DATA_BLOCK DB 701
TITLE = Data to be transmitted to Kongsberg System
VERSION : 0.1


  STRUCT
   PacketNo1 : BYTE ;	// *** TELEGRAM 1 ***   Block 1 (4 Bytes)
   TelegramNo1 : BYTE ;
   TelegramLength1 : WORD ;	//Block 1 End (4 Bytes)
   DG_1_OVERSPEED_TRIP : BOOL ;	//Block 2 (64 Bytes)
   DG_1_FUEL_OIL_PRESSURE : BOOL ;
   DG_1_INJ_FO_PIPE_LEAK_A : BOOL ;
   DG_1_INJ_FO_PIPE_LEAK_B : BOOL ;
   DG_1_LUBE_OIL_LEVEL : BOOL ;
   DG_1_LO_FLT_DIFF_PR : BOOL ;
   DG_1_FO_FLT_DIFF_PR : BOOL ;
   Spare_1_4_7 : BOOL ;
   DG_1_RUNNING : BOOL ;
   DG_1_START_AIR_PRESSURE : BOOL ;
   DG_1_SYMMETRIZATION : BOOL ;
   Spare_1_5_3 : BOOL ;
   Spare_1_5_4 : BOOL ;
   Spare_1_5_5 : BOOL ;
   Spare_1_5_6 : BOOL ;
   Spare_1_5_7 : BOOL ;
   Spare_1_6_0 : BOOL ;
   Spare_1_6_1 : BOOL ;
   Spare_1_6_2 : BOOL ;
   Spare_1_6_3 : BOOL ;
   Spare_1_6_4 : BOOL ;
   Spare_1_6_5 : BOOL ;
   Spare_1_6_6 : BOOL ;
   Spare_1_6_7 : BOOL ;
   Spare_1_7_0 : BOOL ;
   Spare_1_7_1 : BOOL ;
   Spare_1_7_2 : BOOL ;
   Spare_1_7_3 : BOOL ;
   Spare_1_7_4 : BOOL ;
   Spare_1_7_5 : BOOL ;
   Spare_1_7_6 : BOOL ;
   Spare_1_7_7 : BOOL ;
   DG_1_LO_PRESSURE : INT ;
   DG_1_FUEL_OIL_PRESSUREA : INT ;
   DG_1_HT_CW_PRESSURE : INT ;
   DG_1_CA_PRESSURE : INT ;
   DG_1_INJ_COOL_OIL_PRESS : INT ;
   DG_1_RPM : INT ;
   DG_1_TURBO_CHARGER_A_RPM : INT ;
   DG_1_TURBO_CHARGER_B_RPM : INT ;
   DG_1_LO_TEMP : INT ;
   DG_1_COOL_WATER_TEMP : INT ;
   DG_1_CHARG_AIR_TEMP : INT ;
   DG_1_INJ_COOL_OIL_TEMP : INT ;
   DG_1_EXH_GAS_CYL_01_TEMP : INT ;
   DG_1_EXH_GAS_CYL_02_TEMP : INT ;
   DG_1_EXH_GAS_CYL_03_TEMP : INT ;
   DG_1_EXH_GAS_CYL_04_TEMP : INT ;
   DG_1_EXH_GAS_CYL_05_TEMP : INT ;
   DG_1_EXH_GAS_CYL_06_TEMP : INT ;
   DG_1_EXH_GAS_CYL_07_TEMP : INT ;
   DG_1_EXH_GAS_CYL_08_TEMP : INT ;
   DG_1_EXH_GAS_CYL_09_TEMP : INT ;
   DG_1_EXH_GAS_CYL_10_TEMP : INT ;
   DG_1_EXH_GAS_CYL_11_TEMP : INT ;
   DG_1_EXH_GAS_CYL_12_TEMP : INT ;
   DG_1_EXH_GAS_CYL_13_TEMP : INT ;
   DG_1_EXH_GAS_CYL_14_TEMP : INT ;
   DG_1_EXH_GAS_CYL_15_TEMP : INT ;
   DG_1_EXH_GAS_CYL_16_TEMP : INT ;
   DG_1_EXH_CYL_TEMP_MEAN : INT ;
   DG_1_EXH_GAS_TEMP_COMP : INT ;	//Block 2 End (64 Bytes)
   DG_2_OVERSPEED_TRIP : BOOL ;	//Block 3 (64 Bytes)
   DG_2_FUEL_OIL_PRES : BOOL ;
   DG_2_INJ_FO_PIPE_LEAK_A : BOOL ;
   DG_2_INJ_FO_PIPE_LEAK_B : BOOL ;
   DG_2_ENGINE_LUBE_OIL_LVL : BOOL ;
   DG_2_LO_FLT_DIFF_PR : BOOL ;
   DG_2_FO_FLT_DIFF_PR : BOOL ;
   Spare_1_68_7 : BOOL ;
   DG_2_ENGINE_RUNNING : BOOL ;
   DG_2_START_AIR_PRESSURE : BOOL ;
   DG_2_SYMMETRIZATION : BOOL ;
   Spare_1_69_3 : BOOL ;
   Spare_1_69_4 : BOOL ;
   Spare_1_69_5 : BOOL ;
   Spare_1_69_6 : BOOL ;
   Spare_1_69_7 : BOOL ;
   Spare_1_70_0 : BOOL ;
   Spare_1_70_1 : BOOL ;
   Spare_1_70_2 : BOOL ;
   Spare_1_70_3 : BOOL ;
   Spare_1_70_4 : BOOL ;
   Spare_1_70_5 : BOOL ;
   Spare_1_70_6 : BOOL ;
   Spare_1_70_7 : BOOL ;
   Spare_1_71_0 : BOOL ;
   Spare_1_71_1 : BOOL ;
   Spare_1_71_2 : BOOL ;
   Spare_1_71_3 : BOOL ;
   Spare_1_71_4 : BOOL ;
   Spare_1_71_5 : BOOL ;
   Spare_1_71_6 : BOOL ;
   Spare_1_71_7 : BOOL ;
   DG_2_ENGINE_LO_PRESSURE : INT ;
   DG_2_FUEL_OIL_PRESA : INT ;
   DG_2_HT_CW_PRESSURE : INT ;
   DG_2_CA_PRESSURE : INT ;
   DG_2_INJ_COOL_OIL_PRESS : INT ;
   DG_2_ENGINE_RPM : INT ;
   DG_2_TURBO_CHARGER_A_RPM : INT ;
   DG_2_TURBO_CHARGER_B_RPM : INT ;
   DG_2_ENGINE_LO_TEMP : INT ;
   DG_2_COOL_WATER_TEMP : INT ;
   DG_2_CHARG_AIR_TEMP : INT ;
   DG_2_INJ_COOL_OIL_TEMP : INT ;
   DG_2_EXH_GAS_CYL_01_TEMP : INT ;
   DG_2_EXH_GAS_CYL_02_TEMP : INT ;
   DG_2_EXH_GAS_CYL_03_TEMP : INT ;
   DG_2_EXH_GAS_CYL_04_TEMP : INT ;
   DG_2_EXH_GAS_CYL_05_TEMP : INT ;
   DG_2_EXH_GAS_CYL_06_TEMP : INT ;
   DG_2_EXH_GAS_CYL_07_TEMP : INT ;
   DG_2_EXH_GAS_CYL_08_TEMP : INT ;
   DG_2_EXH_GAS_CYL_09_TEMP : INT ;
   DG_2_EXH_GAS_CYL_10_TEMP : INT ;
   DG_2_EXH_GAS_CYL_11_TEMP : INT ;
   DG_2_EXH_GAS_CYL_12_TEMP : INT ;
   DG_2_EXH_GAS_CYL_13_TEMP : INT ;
   DG_2_EXH_GAS_CYL_14_TEMP : INT ;
   DG_2_EXH_GAS_CYL_15_TEMP : INT ;
   DG_2_EXH_GAS_CYL_16_TEMP : INT ;
   DG_2_EXH_CYL_TEMP_MEAN : INT ;
   DG_2_EXH_GAS_TEMP_COMP : INT ;	//Block 3 End (64 Bytes)
   GEN_1_VOLTAGE_L1_L2 : INT ;	//Block 4 (32 Bytes)
   GEN_1_VOLTAGE_L1_L3 : INT ;
   GEN_1_VOLTAGE_L2_L3 : INT ;
   GEN_1_CURRENT_L1_L2 : INT ;
   GEN_1_CURRENT_L1_L3 : INT ;
   GEN_1_CURRENT_L2_L3 : INT ;
   GEN_1_ACTIVE_POWER : INT ;
   GEN_1_POWER_FACTOR : INT ;
   GEN_1_REACTIVE_POWER : INT ;
   GEN_1_WDG_TEMP_L1 : INT ;
   GEN_1_WDG_TEMP_L2 : INT ;
   GEN_1_WDG_TEMP_L3 : INT ;
   GEN_1_BEAR_TEMP_DRIVEEND : INT ;
   GEN_1_BEAR_TEMP_NONDRIVE : INT ;
   GEN_1_COOL_AIR_TEMP : INT ;
   GEN_1_COOL_WATER_TEMP : INT ;	//Block_4_End_(32_Bytes)
   GEN_1_MCB_STATUS : BOOL ;	//Block_5_(4_Bytes)
   GEN_1_MCB_SEC_TO_GND : BOOL ;
   GEN_1_Spare : BOOL ;
   GEN_1_OVER_CURRENT_TRIP : BOOL ;
   GEN_1_REVERSE_POWER_TRIP : BOOL ;
   GEN_1_SHORT_CIRCUIT_TRIP : BOOL ;
   GEN_1_Spare2 : BOOL ;
   GEN_1_DIFF_PROT_TRIP : BOOL ;
   Spare_1_165_0 : BOOL ;
   GEN_1_PREFERENTIAL_TRIP : BOOL ;
   GEN_1_BREAKER_TRIP : BOOL ;
   Spare_1_165_3 : BOOL ;
   GEN_1_PMA_71_FAULT : BOOL ;
   GEN_1_W_LEAK_AIR_COOL : BOOL ;
   Spare_1_165_6 : BOOL ;
   Spare_1_165_7 : BOOL ;
   GEN_1_PMA_71_STATUS : WORD ;	//Block 5 End (4 Bytes)
   GEN_2_VOLTAGE_L1_L2 : INT ;	//Block 6 (32 Bytes)
   GEN_2_VOLTAGE_L1_L3 : INT ;
   GEN_2_VOLTAGE_L2_L3 : INT ;
   GEN_2_CURRENT_L1_L2 : INT ;
   GEN_2_CURRENT_L1_L3 : INT ;
   GEN_2_CURRENT_L2_L3 : INT ;
   GEN_2_ACTIVE_POWER : INT ;
   GEN_2_POWER_FACTOR : INT ;
   GEN_2_REACTIVE_POWER : INT ;
   GEN_2_WDG_TEMP_L1 : INT ;
   GEN_2_WDG_TEMP_L2 : INT ;
   GEN_2_WDG_TEMP_L3 : INT ;
   GEN_2_BEAR_TEMP_DRIVEEND : INT ;
   GEN_2_BEAR_TEMP_NONDRIVE : INT ;
   GEN_2_COOL_AIR_TEMP : INT ;
   GEN_2_COOL_WATER_TEMP : INT ;	//Block 6 End (32 Bytes)
   GEN_2_MCB_STATUS : BOOL ;	//Block 7 (4 Bytes)
   GEN_2_MCB_SEC_TO_GND : BOOL ;
   GEN_2_Spare : BOOL ;
   GEN_2_OVER_CURRENT_TRIP : BOOL ;
   GEN_2_REVERSE_POWER_TRIP : BOOL ;
   GEN_2_SHORT_CIRCUIT_TRIP : BOOL ;
   GEN_2_Spare2 : BOOL ;
   GEN_2_DIFF_PROT_TRIP : BOOL ;
   Spare_1_201_0 : BOOL ;
   GEN_2_PREFERENTIAL_TRIP : BOOL ;
   GEN_2_BREAKER_TRIP : BOOL ;
   Spare_1_201_3 : BOOL ;
   GEN_2_PMA_71_FAULT : BOOL ;
   GEN_2_W_LEAK_AIR_COOL : BOOL ;
   Spare_1_201_6 : BOOL ;
   Spare_1_201_7 : BOOL ;
   GEN_2_PMA_71_STATUS : WORD ;	//Block 7 End (4 Bytes)
   Spare_1_204_0 : BOOL ;	//Block 8 (32 Bytes)
   Spare_1_204_1 : BOOL ;
   Spare_1_204_2 : BOOL ;
   Spare_1_204_3 : BOOL ;
   Spare_1_204_4 : BOOL ;
   Spare_1_204_5 : BOOL ;
   Spare_1_204_6 : BOOL ;
   Spare_1_204_7 : BOOL ;
   Spare_1_205_0 : BOOL ;
   Spare_1_205_1 : BOOL ;
   Spare_1_205_2 : BOOL ;
   Spare_1_205_3 : BOOL ;
   Spare_1_205_4 : BOOL ;
   Spare_1_205_5 : BOOL ;
   Spare_1_205_6 : BOOL ;
   Spare_1_205_7 : BOOL ;
   Spare_1_206_0 : BOOL ;
   Spare_1_206_1 : BOOL ;
   Spare_1_206_2 : BOOL ;
   Spare_1_206_3 : BOOL ;
   Spare_1_206_4 : BOOL ;
   Spare_1_206_5 : BOOL ;
   Spare_1_206_6 : BOOL ;
   Spare_1_206_7 : BOOL ;
   Spare_1_207_0 : BOOL ;
   Spare_1_207_1 : BOOL ;
   Spare_1_207_2 : BOOL ;
   Spare_1_207_3 : BOOL ;
   Spare_1_207_4 : BOOL ;
   Spare_1_207_5 : BOOL ;
   Spare_1_207_6 : BOOL ;
   Spare_1_207_7 : BOOL ;
   Spare_1_208_0 : BOOL ;
   Spare_1_208_1 : BOOL ;
   Spare_1_208_2 : BOOL ;
   Spare_1_208_3 : BOOL ;
   Spare_1_208_4 : BOOL ;
   Spare_1_208_5 : BOOL ;
   Spare_1_208_6 : BOOL ;
   Spare_1_208_7 : BOOL ;
   Spare_1_209_0 : BOOL ;
   Spare_1_209_1 : BOOL ;
   Spare_1_209_2 : BOOL ;
   Spare_1_209_3 : BOOL ;
   Spare_1_209_4 : BOOL ;
   Spare_1_209_5 : BOOL ;
   Spare_1_209_6 : BOOL ;
   Spare_1_209_7 : BOOL ;
   LV_TRANSF_1_WDG_L1_TEMP : INT ;
   LV_TRANSF_1_WDG_L2_TEMP : INT ;
   LV_TRANSF_1_WDG_L3_TEMP : INT ;
   LV_TRANSF_2_WDG_L1_TEMP : INT ;
   LV_TRANSF_2_WDG_L2_TEMP : INT ;
   LV_TRANSF_2_WDG_L3_TEMP : INT ;
   STRT_AIR_PRESS_BOTTLE_1 : INT ;
   STRT_AIR_PRESS_BOTTLE_2 : INT ;
   STRT_AIR_BOT_CAT_PRESS : INT ;
   Spare_1_228 : INT ;
   Spare_1_230 : INT ;
   Spare_1_232 : INT ;
   Spare_1_234 : INT ;	//Block 8 End (32 Bytes)
   PacketNo1B : BYTE ;	//Block 9 (2 Bytes)
   TelegramNo1B : BYTE ;	//Block 9 End (2 Bytes)
   PacketNo2 : BYTE ;	// *** TELEGRAM 2 ***  Block 1 (4 Bytes)
   TelegramNo2 : BYTE ;
   TelegramLength2 : WORD ;	//Block 1 End (4 Bytes)
   DG_3_OVERSPEED_TRIP : BOOL ;	//Block 2 (64 Bytes)
   DG_3_FUEL_OIL_PRESSURE : BOOL ;
   DG_3_INJ_FO_PIPE_LEAK_A : BOOL ;
   DG_3_INJ_FO_PIPE_LEAK_B : BOOL ;
   DG_3_LUBE_OIL_LEVEL : BOOL ;
   DG_3_LO_FLT_DIFF_PR : BOOL ;
   DG_3_FO_FLT_DIFF_PR : BOOL ;
   Spare_2_4_7 : BOOL ;
   DG_3_RUNNING : BOOL ;
   DG_3_START_AIR_PRESSURE : BOOL ;
   DG_3_SYMMETRIZATION : BOOL ;
   Spare_2_5_3 : BOOL ;
   Spare_2_5_4 : BOOL ;
   Spare_2_5_5 : BOOL ;
   Spare_2_5_6 : BOOL ;
   Spare_2_5_7 : BOOL ;
   Spare_2_6_0 : BOOL ;
   Spare_2_6_1 : BOOL ;
   Spare_2_6_2 : BOOL ;
   Spare_2_6_3 : BOOL ;
   Spare_2_6_4 : BOOL ;
   Spare_2_6_5 : BOOL ;
   Spare_2_6_6 : BOOL ;
   Spare_2_6_7 : BOOL ;
   Spare_2_7_0 : BOOL ;
   Spare_2_7_1 : BOOL ;
   Spare_2_7_2 : BOOL ;
   Spare_2_7_3 : BOOL ;
   Spare_2_7_4 : BOOL ;
   Spare_2_7_5 : BOOL ;
   Spare_2_7_6 : BOOL ;
   Spare_2_7_7 : BOOL ;
   DG_3_LO_PRESSURE : INT ;
   DG_3_FUEL_OIL_PRESSUREA : INT ;
   DG_3_HT_CW_PRESSURE : INT ;
   DG_3_CA_PRESSURE : INT ;
   DG_3_INJ_COOL_OIL_PRESS : INT ;
   DG_3_RPM : INT ;
   DG_3_TURBO_CHARGER_A_RPM : INT ;
   DG_3_TURBO_CHARGER_B_RPM : INT ;
   DG_3_LO_TEMP : INT ;
   DG_3_COOL_WATER_TEMP : INT ;
   DG_3_CHARG_AIR_TEMP : INT ;
   DG_3_INJ_COOL_OIL_TEMP : INT ;
   DG_3_EXH_GAS_CYL_01_TEMP : INT ;
   DG_3_EXH_GAS_CYL_02_TEMP : INT ;
   DG_3_EXH_GAS_CYL_03_TEMP : INT ;
   DG_3_EXH_GAS_CYL_04_TEMP : INT ;
   DG_3_EXH_GAS_CYL_05_TEMP : INT ;
   DG_3_EXH_GAS_CYL_06_TEMP : INT ;
   DG_3_EXH_GAS_CYL_07_TEMP : INT ;
   DG_3_EXH_GAS_CYL_08_TEMP : INT ;
   DG_3_EXH_GAS_CYL_09_TEMP : INT ;
   DG_3_EXH_GAS_CYL_10_TEMP : INT ;
   DG_3_EXH_GAS_CYL_11_TEMP : INT ;
   DG_3_EXH_GAS_CYL_12_TEMP : INT ;
   DG_3_EXH_GAS_CYL_13_TEMP : INT ;
   DG_3_EXH_GAS_CYL_14_TEMP : INT ;
   DG_3_EXH_GAS_CYL_15_TEMP : INT ;
   DG_3_EXH_GAS_CYL_16_TEMP : INT ;
   DG_3_EXH_CYL_TEMP_MEAN : INT ;
   DG_3_EXH_GAS_TEMP_COMP : INT ;	//Block 2 End (64 Bytes)
   DG_4_OVERSPEED_TRIP : BOOL ;	//Block 3 (64 Bytes)
   DG_4_FUEL_OIL_PRES : BOOL ;
   DG_4_INJ_FO_PIPE_LEAK_A : BOOL ;
   DG_4_INJ_FO_PIPE_LEAK_B : BOOL ;
   DG_4_ENGINE_LUBE_OIL_LVL : BOOL ;
   DG_4_LO_FLT_DIFF_PR : BOOL ;
   DG_4_FO_FLT_DIFF_PR : BOOL ;
   Spare_2_68_7 : BOOL ;
   DG_4_ENGINE_RUNNING : BOOL ;
   DG_4_START_AIR_PRESSURE : BOOL ;
   DG_4_SYMMETRIZATION : BOOL ;
   Spare_2_69_3 : BOOL ;
   Spare_2_69_4 : BOOL ;
   Spare_2_69_5 : BOOL ;
   Spare_2_69_6 : BOOL ;
   Spare_2_69_7 : BOOL ;
   Spare_2_70_0 : BOOL ;
   Spare_2_70_1 : BOOL ;
   Spare_2_70_2 : BOOL ;
   Spare_2_70_3 : BOOL ;
   Spare_2_70_4 : BOOL ;
   Spare_2_70_5 : BOOL ;
   Spare_2_70_6 : BOOL ;
   Spare_2_70_7 : BOOL ;
   Spare_2_71_0 : BOOL ;
   Spare_2_71_1 : BOOL ;
   Spare_2_71_2 : BOOL ;
   Spare_2_71_3 : BOOL ;
   Spare_2_71_4 : BOOL ;
   Spare_2_71_5 : BOOL ;
   Spare_2_71_6 : BOOL ;
   Spare_2_71_7 : BOOL ;
   DG_4_ENGINE_LO_PRESSURE : INT ;
   DG_4_FUEL_OIL_PRESA : INT ;
   DG_4_HT_CW_PRESSURE : INT ;
   DG_4_CA_PRESSURE : INT ;
   DG_4_INJ_COOL_OIL_PRESS : INT ;
   DG_4_ENGINE_RPM : INT ;
   DG_4_TURBO_CHARGER_A_RPM : INT ;
   DG_4_TURBO_CHARGER_B_RPM : INT ;
   DG_4_ENGINE_LO_TEMP : INT ;
   DG_4_COOL_WATER_TEMP : INT ;
   DG_4_CHARG_AIR_TEMP : INT ;
   DG_4_INJ_COOL_OIL_TEMP : INT ;
   DG_4_EXH_GAS_CYL_01_TEMP : INT ;
   DG_4_EXH_GAS_CYL_02_TEMP : INT ;
   DG_4_EXH_GAS_CYL_03_TEMP : INT ;
   DG_4_EXH_GAS_CYL_04_TEMP : INT ;
   DG_4_EXH_GAS_CYL_05_TEMP : INT ;
   DG_4_EXH_GAS_CYL_06_TEMP : INT ;
   DG_4_EXH_GAS_CYL_07_TEMP : INT ;
   DG_4_EXH_GAS_CYL_08_TEMP : INT ;
   DG_4_EXH_GAS_CYL_09_TEMP : INT ;
   DG_4_EXH_GAS_CYL_10_TEMP : INT ;
   DG_4_EXH_GAS_CYL_11_TEMP : INT ;
   DG_4_EXH_GAS_CYL_12_TEMP : INT ;
   DG_4_EXH_GAS_CYL_13_TEMP : INT ;
   DG_4_EXH_GAS_CYL_14_TEMP : INT ;
   DG_4_EXH_GAS_CYL_15_TEMP : INT ;
   DG_4_EXH_GAS_CYL_16_TEMP : INT ;
   DG_4_EXH_CYL_TEMP_MEAN : INT ;
   DG_4_EXH_GAS_TEMP_COMP : INT ;	//Block 3 End (64 Bytes)
   GEN_3_VOLTAGE_L1_L2 : INT ;	//Block 4 (32 Bytes)
   GEN_3_VOLTAGE_L1_L3 : INT ;
   GEN_3_VOLTAGE_L2_L3 : INT ;
   GEN_3_CURRENT_L1_L2 : INT ;
   GEN_3_CURRENT_L1_L3 : INT ;
   GEN_3_CURRENT_L2_L3 : INT ;
   GEN_3_ACTIVE_POWER : INT ;
   GEN_3_POWER_FACTOR : INT ;
   GEN_3_REACTIVE_POWER : INT ;
   GEN_3_WDG_TEMP_L1 : INT ;
   GEN_3_WDG_TEMP_L2 : INT ;
   GEN_3_WDG_TEMP_L3 : INT ;
   GEN_3_BEAR_TEMP_DRIVEEND : INT ;
   GEN_3_BEAR_TEMP_NONDRIVE : INT ;
   GEN_3_COOL_AIR_TEMP : INT ;
   GEN_3_COOL_WATER_TEMP : INT ;	//Block_4_End_(32_Bytes)
   GEN_3_MCB_STATUS : BOOL ;	//Block_5_(4_Bytes)
   GEN_3_MCB_SEC_TO_GND : BOOL ;
   GEN_3_Spare : BOOL ;
   GEN_3_OVER_CURRENT_TRIP : BOOL ;
   GEN_3_REVERSE_POWER_TRIP : BOOL ;
   GEN_3_SHORT_CIRCUIT_TRIP : BOOL ;
   GEN_3_Spare2 : BOOL ;
   GEN_3_DIFF_PROT_TRIP : BOOL ;
   Spare_2_165_0 : BOOL ;
   GEN_3_PREFERENTIAL_TRIP : BOOL ;
   GEN_3_BREAKER_TRIP : BOOL ;
   Spare_2_165_3 : BOOL ;
   GEN_3_PMA_71_FAULT : BOOL ;
   GEN_3_W_LEAK_AIR_COOL : BOOL ;
   Spare_2_165_6 : BOOL ;
   Spare_2_165_7 : BOOL ;
   GEN_3_PMA_71_STATUS : WORD ;	//Block 5 End (4 Bytes)
   GEN_4_VOLTAGE_L1_L2 : INT ;	//Block 6 (32 Bytes)
   GEN_4_VOLTAGE_L1_L3 : INT ;
   GEN_4_VOLTAGE_L2_L3 : INT ;
   GEN_4_CURRENT_L1_L2 : INT ;
   GEN_4_CURRENT_L1_L3 : INT ;
   GEN_4_CURRENT_L2_L3 : INT ;
   GEN_4_ACTIVE_POWER : INT ;
   GEN_4_POWER_FACTOR : INT ;
   GEN_4_REACTIVE_POWER : INT ;
   GEN_4_WDG_TEMP_L1 : INT ;
   GEN_4_WDG_TEMP_L2 : INT ;
   GEN_4_WDG_TEMP_L3 : INT ;
   GEN_4_BEAR_TEMP_DRIVEEND : INT ;
   GEN_4_BEAR_TEMP_NONDRIVE : INT ;
   GEN_4_COOL_AIR_TEMP : INT ;
   GEN_4_COOL_WATER_TEMP : INT ;	//Block 6 End (32 Bytes)
   GEN_4_MCB_STATUS : BOOL ;	//Block 7 (4 Bytes)
   GEN_4_MCB_SEC_TO_GND : BOOL ;
   GEN_4_Spare : BOOL ;
   GEN_4_OVER_CURRENT_TRIP : BOOL ;
   GEN_4_REVERSE_POWER_TRIP : BOOL ;
   GEN_4_SHORT_CIRCUIT_TRIP : BOOL ;
   GEN_4_Spare2 : BOOL ;
   GEN_4_DIFF_PROT_TRIP : BOOL ;
   Spare_2_201_0 : BOOL ;
   GEN_4_PREFERENTIAL_TRIP : BOOL ;
   GEN_4_BREAKER_TRIP : BOOL ;
   Spare_2_201_3 : BOOL ;
   GEN_4_PMA_71_FAULT : BOOL ;
   GEN_4_W_LEAK_AIR_COOL : BOOL ;
   Spare_2_201_6 : BOOL ;
   Spare_2_201_7 : BOOL ;
   GEN_4_PMA_71_STATUS : WORD ;	//Block 7 End (4 Bytes)
   Spare_2_204_0 : BOOL ;	//Block 8 (32 Bytes)
   Spare_2_204_1 : BOOL ;
   Spare_2_204_2 : BOOL ;
   Spare_2_204_3 : BOOL ;
   Spare_2_204_4 : BOOL ;
   Spare_2_204_5 : BOOL ;
   Spare_2_204_6 : BOOL ;
   Spare_2_204_7 : BOOL ;
   Spare_2_205_0 : BOOL ;
   Spare_2_205_1 : BOOL ;
   Spare_2_205_2 : BOOL ;
   Spare_2_205_3 : BOOL ;
   Spare_2_205_4 : BOOL ;
   Spare_2_205_5 : BOOL ;
   Spare_2_205_6 : BOOL ;
   Spare_2_205_7 : BOOL ;
   Spare_2_206_0 : BOOL ;
   Spare_2_206_1 : BOOL ;
   Spare_2_206_2 : BOOL ;
   Spare_2_206_3 : BOOL ;
   Spare_2_206_4 : BOOL ;
   Spare_2_206_5 : BOOL ;
   Spare_2_206_6 : BOOL ;
   Spare_2_206_7 : BOOL ;
   Spare_2_207_0 : BOOL ;
   Spare_2_207_1 : BOOL ;
   Spare_2_207_2 : BOOL ;
   Spare_2_207_3 : BOOL ;
   Spare_2_207_4 : BOOL ;
   Spare_2_207_5 : BOOL ;
   Spare_2_207_6 : BOOL ;
   Spare_2_207_7 : BOOL ;
   Spare_2_208_0 : BOOL ;
   Spare_2_208_1 : BOOL ;
   Spare_2_208_2 : BOOL ;
   Spare_2_208_3 : BOOL ;
   Spare_2_208_4 : BOOL ;
   Spare_2_208_5 : BOOL ;
   Spare_2_208_6 : BOOL ;
   Spare_2_208_7 : BOOL ;
   Spare_2_209_0 : BOOL ;
   Spare_2_209_1 : BOOL ;
   Spare_2_209_2 : BOOL ;
   Spare_2_209_3 : BOOL ;
   Spare_2_209_4 : BOOL ;
   Spare_2_209_5 : BOOL ;
   Spare_2_209_6 : BOOL ;
   Spare_2_209_7 : BOOL ;
   Spare_2_210 : INT ;
   Spare_2_212 : INT ;
   Spare_2_214 : INT ;
   Spare_2_216 : INT ;
   Spare_2_218 : INT ;
   Spare_2_220 : INT ;
   Spare_2_222 : INT ;
   Spare_2_224 : INT ;
   Spare_2_226 : INT ;
   Spare_2_228 : INT ;
   Spare_2_230 : INT ;
   Spare_2_232 : INT ;
   Spare_2_234 : INT ;	//Block 8 End (32 Bytes)
   PacketNo2B : BYTE ;	//Block 9 (2 Bytes)
   TelegramNo2B : BYTE ;	//Block 9 End (2 Bytes)
   PacketNo3 : BYTE ;	// *** TELEGRAM 3 ***  Block 1 (4 Bytes)
   TelegramNo3 : BYTE ;
   TelegramLength3 : WORD ;	//Block 1 End (4 Bytes)
   DG_5_OVERSPEED_TRIP : BOOL ;	//Block 2 (64 Bytes)
   DG_5_FUEL_OIL_PRESSURE : BOOL ;
   DG_5_INJ_FO_PIPE_LEAK_A : BOOL ;
   DG_5_INJ_FO_PIPE_LEAK_B : BOOL ;
   DG_5_LUBE_OIL_LEVEL : BOOL ;
   DG_5_LO_FLT_DIFF_PR : BOOL ;
   DG_5_FO_FLT_DIFF_PR : BOOL ;
   Spare_3_4_7 : BOOL ;
   DG_5_RUNNING : BOOL ;
   DG_5_START_AIR_PRESSURE : BOOL ;
   DG_5_SYMMETRIZATION : BOOL ;
   Spare_3_5_3 : BOOL ;
   Spare_3_5_4 : BOOL ;
   Spare_3_5_5 : BOOL ;
   Spare_3_5_6 : BOOL ;
   Spare_3_5_7 : BOOL ;
   Spare_3_6_0 : BOOL ;
   Spare_3_6_1 : BOOL ;
   Spare_3_6_2 : BOOL ;
   Spare_3_6_3 : BOOL ;
   Spare_3_6_4 : BOOL ;
   Spare_3_6_5 : BOOL ;
   Spare_3_6_6 : BOOL ;
   Spare_3_6_7 : BOOL ;
   Spare_3_7_0 : BOOL ;
   Spare_3_7_1 : BOOL ;
   Spare_3_7_2 : BOOL ;
   Spare_3_7_3 : BOOL ;
   Spare_3_7_4 : BOOL ;
   Spare_3_7_5 : BOOL ;
   Spare_3_7_6 : BOOL ;
   Spare_3_7_7 : BOOL ;
   DG_5_LO_PRESSURE : INT ;
   DG_5_FUEL_OIL_PRESSUREA : INT ;
   DG_5_HT_CW_PRESSURE : INT ;
   DG_5_CA_PRESSURE : INT ;
   DG_5_INJ_COOL_OIL_PRESS : INT ;
   DG_5_RPM : INT ;
   DG_5_TURBO_CHARGER_A_RPM : INT ;
   DG_5_TURBO_CHARGER_B_RPM : INT ;
   DG_5_LO_TEMP : INT ;
   DG_5_COOL_WATER_TEMP : INT ;
   DG_5_CHARG_AIR_TEMP : INT ;
   DG_5_INJ_COOL_OIL_TEMP : INT ;
   DG_5_EXH_GAS_CYL_01_TEMP : INT ;
   DG_5_EXH_GAS_CYL_02_TEMP : INT ;
   DG_5_EXH_GAS_CYL_03_TEMP : INT ;
   DG_5_EXH_GAS_CYL_04_TEMP : INT ;
   DG_5_EXH_GAS_CYL_05_TEMP : INT ;
   DG_5_EXH_GAS_CYL_06_TEMP : INT ;
   DG_5_EXH_GAS_CYL_07_TEMP : INT ;
   DG_5_EXH_GAS_CYL_08_TEMP : INT ;
   DG_5_EXH_GAS_CYL_09_TEMP : INT ;
   DG_5_EXH_GAS_CYL_10_TEMP : INT ;
   DG_5_EXH_GAS_CYL_11_TEMP : INT ;
   DG_5_EXH_GAS_CYL_12_TEMP : INT ;
   DG_5_EXH_GAS_CYL_13_TEMP : INT ;
   DG_5_EXH_GAS_CYL_14_TEMP : INT ;
   DG_5_EXH_GAS_CYL_15_TEMP : INT ;
   DG_5_EXH_GAS_CYL_16_TEMP : INT ;
   DG_5_EXH_CYL_TEMP_MEAN : INT ;
   DG_5_EXH_GAS_TEMP_COMP : INT ;	//Block 2 End (64 Bytes)
   DG_6_OVERSPEED_TRIP : BOOL ;	//Block 3 (64 Bytes)
   DG_6_FUEL_OIL_PRES : BOOL ;
   DG_6_INJ_FO_PIPE_LEAK_A : BOOL ;
   DG_6_INJ_FO_PIPE_LEAK_B : BOOL ;
   DG_6_ENGINE_LUBE_OIL_LVL : BOOL ;
   DG_6_LO_FLT_DIFF_PR : BOOL ;
   DG_6_FO_FLT_DIFF_PR : BOOL ;
   Spare_3_68_7 : BOOL ;
   DG_6_ENGINE_RUNNING : BOOL ;
   DG_6_START_AIR_PRESSURE : BOOL ;
   DG_6_SYMMETRIZATION : BOOL ;
   Spare_3_69_3 : BOOL ;
   Spare_3_69_4 : BOOL ;
   Spare_3_69_5 : BOOL ;
   Spare_3_69_6 : BOOL ;
   Spare_3_69_7 : BOOL ;
   Spare_3_70_0 : BOOL ;
   Spare_3_70_1 : BOOL ;
   Spare_3_70_2 : BOOL ;
   Spare_3_70_3 : BOOL ;
   Spare_3_70_4 : BOOL ;
   Spare_3_70_5 : BOOL ;
   Spare_3_70_6 : BOOL ;
   Spare_3_70_7 : BOOL ;
   Spare_3_71_0 : BOOL ;
   Spare_3_71_1 : BOOL ;
   Spare_3_71_2 : BOOL ;
   Spare_3_71_3 : BOOL ;
   Spare_3_71_4 : BOOL ;
   Spare_3_71_5 : BOOL ;
   Spare_3_71_6 : BOOL ;
   Spare_3_71_7 : BOOL ;
   DG_6_ENGINE_LO_PRESSURE : INT ;
   DG_6_FUEL_OIL_PRESA : INT ;
   DG_6_HT_CW_PRESSURE : INT ;
   DG_6_CA_PRESSURE : INT ;
   DG_6_INJ_COOL_OIL_PRESS : INT ;
   DG_6_ENGINE_RPM : INT ;
   DG_6_TURBO_CHARGER_A_RPM : INT ;
   DG_6_TURBO_CHARGER_B_RPM : INT ;
   DG_6_ENGINE_LO_TEMP : INT ;
   DG_6_COOL_WATER_TEMP : INT ;
   DG_6_CHARG_AIR_TEMP : INT ;
   DG_6_INJ_COOL_OIL_TEMP : INT ;
   DG_6_EXH_GAS_CYL_01_TEMP : INT ;
   DG_6_EXH_GAS_CYL_02_TEMP : INT ;
   DG_6_EXH_GAS_CYL_03_TEMP : INT ;
   DG_6_EXH_GAS_CYL_04_TEMP : INT ;
   DG_6_EXH_GAS_CYL_05_TEMP : INT ;
   DG_6_EXH_GAS_CYL_06_TEMP : INT ;
   DG_6_EXH_GAS_CYL_07_TEMP : INT ;
   DG_6_EXH_GAS_CYL_08_TEMP : INT ;
   DG_6_EXH_GAS_CYL_09_TEMP : INT ;
   DG_6_EXH_GAS_CYL_10_TEMP : INT ;
   DG_6_EXH_GAS_CYL_11_TEMP : INT ;
   DG_6_EXH_GAS_CYL_12_TEMP : INT ;
   DG_6_EXH_GAS_CYL_13_TEMP : INT ;
   DG_6_EXH_GAS_CYL_14_TEMP : INT ;
   DG_6_EXH_GAS_CYL_15_TEMP : INT ;
   DG_6_EXH_GAS_CYL_16_TEMP : INT ;
   DG_6_EXH_CYL_TEMP_MEAN : INT ;
   DG_6_EXH_GAS_TEMP_COMP : INT ;	//Block 3 End (64 Bytes)
   GEN_5_VOLTAGE_L1_L2 : INT ;	//Block 4 (32 Bytes)
   GEN_5_VOLTAGE_L1_L3 : INT ;
   GEN_5_VOLTAGE_L2_L3 : INT ;
   GEN_5_CURRENT_L1_L2 : INT ;
   GEN_5_CURRENT_L1_L3 : INT ;
   GEN_5_CURRENT_L2_L3 : INT ;
   GEN_5_ACTIVE_POWER : INT ;
   GEN_5_POWER_FACTOR : INT ;
   GEN_5_REACTIVE_POWER : INT ;
   GEN_5_WDG_TEMP_L1 : INT ;
   GEN_5_WDG_TEMP_L2 : INT ;
   GEN_5_WDG_TEMP_L3 : INT ;
   GEN_5_BEAR_TEMP_DRIVEEND : INT ;
   GEN_5_BEAR_TEMP_NONDRIVE : INT ;
   GEN_5_COOL_AIR_TEMP : INT ;
   GEN_5_COOL_WATER_TEMP : INT ;	//Block_4_End_(32_Bytes)
   GEN_5_MCB_STATUS : BOOL ;	//Block_5_(4_Bytes)
   GEN_5_MCB_SEC_TO_GND : BOOL ;
   GEN_5_Spare : BOOL ;
   GEN_5_OVER_CURRENT_TRIP : BOOL ;
   GEN_5_REVERSE_POWER_TRIP : BOOL ;
   GEN_5_SHORT_CIRCUIT_TRIP : BOOL ;
   GEN_5_Spare2 : BOOL ;
   GEN_5_DIFF_PROT_TRIP : BOOL ;
   Spare_3_165_0 : BOOL ;
   GEN_5_PREFERENTIAL_TRIP : BOOL ;
   GEN_5_BREAKER_TRIP : BOOL ;
   Spare_3_165_3 : BOOL ;
   GEN_5_PMA_71_FAULT : BOOL ;
   GEN_5_W_LEAK_AIR_COOL : BOOL ;
   Spare_3_165_6 : BOOL ;
   Spare_3_165_7 : BOOL ;
   GEN_5_PMA_71_STATUS : WORD ;	//Block 5 End (4 Bytes)
   GEN_6_VOLTAGE_L1_L2 : INT ;	//Block 6 (32 Bytes)
   GEN_6_VOLTAGE_L1_L3 : INT ;
   GEN_6_VOLTAGE_L2_L3 : INT ;
   GEN_6_CURRENT_L1_L2 : INT ;
   GEN_6_CURRENT_L1_L3 : INT ;
   GEN_6_CURRENT_L2_L3 : INT ;
   GEN_6_ACTIVE_POWER : INT ;
   GEN_6_POWER_FACTOR : INT ;
   GEN_6_REACTIVE_POWER : INT ;
   GEN_6_WDG_TEMP_L1 : INT ;
   GEN_6_WDG_TEMP_L2 : INT ;
   GEN_6_WDG_TEMP_L3 : INT ;
   GEN_6_BEAR_TEMP_DRIVEEND : INT ;
   GEN_6_BEAR_TEMP_NONDRIVE : INT ;
   GEN_6_COOL_AIR_TEMP : INT ;
   GEN_6_COOL_WATER_TEMP : INT ;	//Block 6 End (32 Bytes)
   GEN_6_MCB_STATUS : BOOL ;	//Block 7 (4 Bytes)
   GEN_6_MCB_SEC_TO_GND : BOOL ;
   GEN_6_Spare : BOOL ;
   GEN_6_OVER_CURRENT_TRIP : BOOL ;
   GEN_6_REVERSE_POWER_TRIP : BOOL ;
   GEN_6_SHORT_CIRCUIT_TRIP : BOOL ;
   GEN_6_Spare2 : BOOL ;
   GEN_6_DIFF_PROT_TRIP : BOOL ;
   Spare_3_201_0 : BOOL ;
   GEN_6_PREFERENTIAL_TRIP : BOOL ;
   GEN_6_BREAKER_TRIP : BOOL ;
   Spare_3_201_3 : BOOL ;
   GEN_6_PMA_71_FAULT : BOOL ;
   GEN_6_W_LEAK_AIR_COOL : BOOL ;
   Spare_3_201_6 : BOOL ;
   Spare_3_201_7 : BOOL ;
   GEN_6_PMA_71_STATUS : WORD ;	//Block 7 End (4 Bytes)
   Spare_3_204_0 : BOOL ;	//Block 8 (32 Bytes)
   Spare_3_204_1 : BOOL ;
   Spare_3_204_2 : BOOL ;
   Spare_3_204_3 : BOOL ;
   Spare_3_204_4 : BOOL ;
   Spare_3_204_5 : BOOL ;
   Spare_3_204_6 : BOOL ;
   Spare_3_204_7 : BOOL ;
   Spare_3_205_0 : BOOL ;
   Spare_3_205_1 : BOOL ;
   Spare_3_205_2 : BOOL ;
   Spare_3_205_3 : BOOL ;
   Spare_3_205_4 : BOOL ;
   Spare_3_205_5 : BOOL ;
   Spare_3_205_6 : BOOL ;
   Spare_3_205_7 : BOOL ;
   Spare_3_206_0 : BOOL ;
   Spare_3_206_1 : BOOL ;
   Spare_3_206_2 : BOOL ;
   Spare_3_206_3 : BOOL ;
   Spare_3_206_4 : BOOL ;
   Spare_3_206_5 : BOOL ;
   Spare_3_206_6 : BOOL ;
   Spare_3_206_7 : BOOL ;
   Spare_3_207_0 : BOOL ;
   Spare_3_207_1 : BOOL ;
   Spare_3_207_2 : BOOL ;
   Spare_3_207_3 : BOOL ;
   Spare_3_207_4 : BOOL ;
   Spare_3_207_5 : BOOL ;
   Spare_3_207_6 : BOOL ;
   Spare_3_207_7 : BOOL ;
   Spare_3_208_0 : BOOL ;
   Spare_3_208_1 : BOOL ;
   Spare_3_208_2 : BOOL ;
   Spare_3_208_3 : BOOL ;
   Spare_3_208_4 : BOOL ;
   Spare_3_208_5 : BOOL ;
   Spare_3_208_6 : BOOL ;
   Spare_3_208_7 : BOOL ;
   Spare_3_209_0 : BOOL ;
   Spare_3_209_1 : BOOL ;
   Spare_3_209_2 : BOOL ;
   Spare_3_209_3 : BOOL ;
   Spare_3_209_4 : BOOL ;
   Spare_3_209_5 : BOOL ;
   Spare_3_209_6 : BOOL ;
   Spare_3_209_7 : BOOL ;
   Spare_3_210 : INT ;
   Spare_3_212 : INT ;
   Spare_3_214 : INT ;
   Spare_3_216 : INT ;
   Spare_3_218 : INT ;
   Spare_3_220 : INT ;
   Spare_3_222 : INT ;
   Spare_3_224 : INT ;
   Spare_3_226 : INT ;
   Spare_3_228 : INT ;
   Spare_3_230 : INT ;
   Spare_3_232 : INT ;
   Spare_3_234 : INT ;	//Block 8 End (32 Bytes)
   PacketNo3B : BYTE ;	//Block 9 (2 Bytes)
   TelegramNo3B : BYTE ;	//Block 9 End (2 Bytes)
   PacketNo4 : BYTE ;	// *** TELEGRAM 4 ***  Block 1 (4 Bytes)
   TelegramNo4 : BYTE ;
   TelegramLength4 : WORD ;	//Block 1 End (4 Bytes)
   DG_7_ENG_COOL_LVL : BOOL ;	//Block 2 (64 Bytes)
   DG_7_ENG_LO_PRESS : BOOL ;
   DG_7_FO_FLT_DIFF_PR : BOOL ;
   DG_7_LO_FLT_DIFF_PR : BOOL ;
   DG_7_ENG_CRK_CASE_PR : BOOL ;
   DG_7_MAR_GEAR_OIL_PR : BOOL ;
   DG_7_ENG_JACK_WT_TEMP_HI : BOOL ;
   DG_7_ENG_JACK_WT_TEMP_LO : BOOL ;
   DG_7_ENG_EXH_GAS_TEMP : BOOL ;
   DG_7_ENG_AFT_COOL_TEMP : BOOL ;
   DG_7_MAR_GEAR_OIL_TEMP : BOOL ;
   DG_7_ENG_OVERSPEED : BOOL ;
   DG_7_EL_FUEL_INJ : BOOL ;
   DG_7_ENG_AIR_RESTR : BOOL ;
   DG_7_SYMMETRIZATION : BOOL ;
   Spare_4_5_7 : BOOL ;
   Spare_4_6_0 : BOOL ;
   Spare_4_6_1 : BOOL ;
   Spare_4_6_2 : BOOL ;
   Spare_4_6_3 : BOOL ;
   Spare_4_6_4 : BOOL ;
   Spare_4_6_5 : BOOL ;
   Spare_4_6_6 : BOOL ;
   Spare_4_6_7 : BOOL ;
   Spare_4_7_0 : BOOL ;
   Spare_4_7_1 : BOOL ;
   Spare_4_7_2 : BOOL ;
   Spare_4_7_3 : BOOL ;
   Spare_4_7_4 : BOOL ;
   Spare_4_7_5 : BOOL ;
   Spare_4_7_6 : BOOL ;
   Spare_4_7_7 : BOOL ;
   Spare_4_8 : INT ;
   Spare_4_10 : INT ;
   Spare_4_12 : INT ;
   Spare_4_14 : INT ;
   Spare_4_16 : INT ;
   Spare_4_18 : INT ;
   Spare_4_20 : INT ;
   Spare_4_22 : INT ;
   Spare_4_24 : INT ;
   Spare_4_26 : INT ;
   Spare_4_28 : INT ;
   Spare_4_30 : INT ;
   DG_7_EXH_GAS_CYL_01_TEMP : INT ;
   DG_7_EXH_GAS_CYL_02_TEMP : INT ;
   DG_7_EXH_GAS_CYL_03_TEMP : INT ;
   DG_7_EXH_GAS_CYL_04_TEMP : INT ;
   DG_7_EXH_GAS_CYL_05_TEMP : INT ;
   DG_7_EXH_GAS_CYL_06_TEMP : INT ;
   DG_7_EXH_GAS_CYL_07_TEMP : INT ;
   DG_7_EXH_GAS_CYL_08_TEMP : INT ;
   DG_7_EXH_GAS_CYL_09_TEMP : INT ;
   DG_7_EXH_GAS_CYL_10_TEMP : INT ;
   DG_7_EXH_GAS_CYL_11_TEMP : INT ;
   DG_7_EXH_GAS_CYL_12_TEMP : INT ;
   DG_7_EXH_GAS_CYL_13_TEMP : INT ;
   DG_7_EXH_GAS_CYL_14_TEMP : INT ;
   DG_7_EXH_GAS_CYL_15_TEMP : INT ;
   DG_7_EXH_GAS_CYL_16_TEMP : INT ;
   DG_7_EXH_CYL_TEMP_MEAN : INT ;
   DG_7_EXH_GAS_TEMP_COMP : INT ;	//Block 2 End (64 Bytes)
   DG_8_ENG_COOL_LVL : BOOL ;	//Block 3 (64 Bytes)
   DG_8_ENG_LO_PRESS : BOOL ;
   DG_8_FO_FLT_DIFF_PR : BOOL ;
   DG_8_LO_FLT_DIFF_PR : BOOL ;
   DG_8_ENG_CRK_CASE_PR : BOOL ;
   DG_8_MAR_GEAR_OIL_PR : BOOL ;
   DG_8_ENG_JACK_WT_TEMP_HI : BOOL ;
   DG_8_ENG_JACK_WT_TEMP_LO : BOOL ;
   DG_8_ENG_EXH_GAS_TEMP : BOOL ;
   DG_8_ENG_AFT_COOL_TEMP : BOOL ;
   DG_8_MAR_GEAR_OIL_TEMP : BOOL ;
   DG_8_ENG_OVERSPEED : BOOL ;
   DG_8_EL_FUEL_INJ : BOOL ;
   DG_8_ENG_AIR_RESTR : BOOL ;
   DG_8_SYMMETRIZATION : BOOL ;
   Spare_4_69_7 : BOOL ;
   Spare_4_70_0 : BOOL ;
   Spare_4_70_1 : BOOL ;
   Spare_4_70_2 : BOOL ;
   Spare_4_70_3 : BOOL ;
   Spare_4_70_4 : BOOL ;
   Spare_4_70_5 : BOOL ;
   Spare_4_70_6 : BOOL ;
   Spare_4_70_7 : BOOL ;
   Spare_4_71_0 : BOOL ;
   Spare_4_71_1 : BOOL ;
   Spare_4_71_2 : BOOL ;
   Spare_4_71_3 : BOOL ;
   Spare_4_71_4 : BOOL ;
   Spare_4_71_5 : BOOL ;
   Spare_4_71_6 : BOOL ;
   Spare_4_71_7 : BOOL ;
   Spare_4_72 : INT ;
   Spare_4_74 : INT ;
   Spare_4_76 : INT ;
   Spare_4_78 : INT ;
   Spare_4_80 : INT ;
   Spare_4_82 : INT ;
   Spare_4_84 : INT ;
   Spare_4_86 : INT ;
   Spare_4_88 : INT ;
   Spare_4_90 : INT ;
   Spare_4_92 : INT ;
   Spare_4_94 : INT ;
   DG_8_EXH_GAS_CYL_01_TEMP : INT ;
   DG_8_EXH_GAS_CYL_02_TEMP : INT ;
   DG_8_EXH_GAS_CYL_03_TEMP : INT ;
   DG_8_EXH_GAS_CYL_04_TEMP : INT ;
   DG_8_EXH_GAS_CYL_05_TEMP : INT ;
   DG_8_EXH_GAS_CYL_06_TEMP : INT ;
   DG_8_EXH_GAS_CYL_07_TEMP : INT ;
   DG_8_EXH_GAS_CYL_08_TEMP : INT ;
   DG_8_EXH_GAS_CYL_09_TEMP : INT ;
   DG_8_EXH_GAS_CYL_10_TEMP : INT ;
   DG_8_EXH_GAS_CYL_11_TEMP : INT ;
   DG_8_EXH_GAS_CYL_12_TEMP : INT ;
   DG_8_EXH_GAS_CYL_13_TEMP : INT ;
   DG_8_EXH_GAS_CYL_14_TEMP : INT ;
   DG_8_EXH_GAS_CYL_15_TEMP : INT ;
   DG_8_EXH_GAS_CYL_16_TEMP : INT ;
   DG_8_EXH_CYL_TEMP_MEAN : INT ;
   DG_8_EXH_GAS_TEMP_COMP : INT ;	//Block 3 End (64 Bytes)
   GEN_7_VOLTAGE_L1_L2 : INT ;	//Block 4 (32 Bytes)
   GEN_7_VOLTAGE_L1_L3 : INT ;
   GEN_7_VOLTAGE_L2_L3 : INT ;
   GEN_7_CURRENT_L1_L2 : INT ;
   GEN_7_CURRENT_L1_L3 : INT ;
   GEN_7_CURRENT_L2_L3 : INT ;
   GEN_7_ACTIVE_POWER : INT ;
   GEN_7_POWER_FACTOR : INT ;
   GEN_7_REACTIVE_POWER : INT ;
   GEN_7_WDG_TEMP_L1 : INT ;
   GEN_7_WDG_TEMP_L2 : INT ;
   GEN_7_WDG_TEMP_L3 : INT ;
   GEN_7_BEAR_TEMP_DRIVEEND : INT ;
   GEN_7_BEAR_TEMP_NONDRIVE : INT ;
   GEN_7_COOL_AIR_TEMP : INT ;
   GEN_7_COOL_WATER_TEMP : INT ;	//Block_4_End_(32_Bytes)
   GEN_7_MCB_STATUS : BOOL ;	//Block_5_(4_Bytes)
   GEN_7_MCB_SEC_TO_GND : BOOL ;
   GEN_7_Spare : BOOL ;
   GEN_7_OVER_CURRENT_TRIP : BOOL ;
   GEN_7_REVERSE_POWER_TRIP : BOOL ;
   GEN_7_SHORT_CIRCUIT_TRIP : BOOL ;
   GEN_7_Spare2 : BOOL ;
   GEN_7_DIFF_PROT_TRIP : BOOL ;
   Spare_4_165_0 : BOOL ;
   GEN_7_PREFERENTIAL_TRIP : BOOL ;
   GEN_7_BREAKER_TRIP : BOOL ;
   Spare_4_165_3 : BOOL ;
   GEN_7_PMA_71_FAULT : BOOL ;
   GEN_7_W_LEAK_AIR_COOL : BOOL ;
   Spare_4_165_6 : BOOL ;
   Spare_4_165_7 : BOOL ;
   GEN_7_PMA_71_STATUS : WORD ;	//Block 5 End (4 Bytes)
   GEN_8_VOLTAGE_L1_L2 : INT ;	//Block 6 (32 Bytes)
   GEN_8_VOLTAGE_L1_L3 : INT ;
   GEN_8_VOLTAGE_L2_L3 : INT ;
   GEN_8_CURRENT_L1_L2 : INT ;
   GEN_8_CURRENT_L1_L3 : INT ;
   GEN_8_CURRENT_L2_L3 : INT ;
   GEN_8_ACTIVE_POWER : INT ;
   GEN_8_POWER_FACTOR : INT ;
   GEN_8_REACTIVE_POWER : INT ;
   GEN_8_WDG_TEMP_L1 : INT ;
   GEN_8_WDG_TEMP_L2 : INT ;
   GEN_8_WDG_TEMP_L3 : INT ;
   GEN_8_BEAR_TEMP_DRIVEEND : INT ;
   GEN_8_BEAR_TEMP_NONDRIVE : INT ;
   GEN_8_COOL_AIR_TEMP : INT ;
   GEN_8_COOL_WATER_TEMP : INT ;	//Block 6 End (32 Bytes)
   GEN_8_MCB_STATUS : BOOL ;	//Block 7 (4 Bytes)
   GEN_8_MCB_SEC_TO_GND : BOOL ;
   GEN_8_Spare : BOOL ;
   GEN_8_OVER_CURRENT_TRIP : BOOL ;
   GEN_8_REVERSE_POWER_TRIP : BOOL ;
   GEN_8_SHORT_CIRCUIT_TRIP : BOOL ;
   GEN_8_Spare2 : BOOL ;
   GEN_8_DIFF_PROT_TRIP : BOOL ;
   Spare_4_201_0 : BOOL ;
   GEN_8_PREFERENTIAL_TRIP : BOOL ;
   GEN_8_BREAKER_TRIP : BOOL ;
   Spare_4_201_3 : BOOL ;
   GEN_8_PMA_71_FAULT : BOOL ;
   GEN_8_W_LEAK_AIR_COOL : BOOL ;
   Spare_4_201_6 : BOOL ;
   Spare_4_201_7 : BOOL ;
   GEN_8_PMA_71_STATUS : WORD ;	//Block 7 End (4 Bytes)
   Spare_4_204_0 : BOOL ;	//Block 8 (32 Bytes)
   Spare_4_204_1 : BOOL ;
   Spare_4_204_2 : BOOL ;
   Spare_4_204_3 : BOOL ;
   Spare_4_204_4 : BOOL ;
   Spare_4_204_5 : BOOL ;
   Spare_4_204_6 : BOOL ;
   Spare_4_204_7 : BOOL ;
   Spare_4_205_0 : BOOL ;
   Spare_4_205_1 : BOOL ;
   Spare_4_205_2 : BOOL ;
   Spare_4_205_3 : BOOL ;
   Spare_4_205_4 : BOOL ;
   Spare_4_205_5 : BOOL ;
   Spare_4_205_6 : BOOL ;
   Spare_4_205_7 : BOOL ;
   Spare_4_206_0 : BOOL ;
   Spare_4_206_1 : BOOL ;
   Spare_4_206_2 : BOOL ;
   Spare_4_206_3 : BOOL ;
   Spare_4_206_4 : BOOL ;
   Spare_4_206_5 : BOOL ;
   Spare_4_206_6 : BOOL ;
   Spare_4_206_7 : BOOL ;
   Spare_4_207_0 : BOOL ;
   Spare_4_207_1 : BOOL ;
   Spare_4_207_2 : BOOL ;
   Spare_4_207_3 : BOOL ;
   Spare_4_207_4 : BOOL ;
   Spare_4_207_5 : BOOL ;
   Spare_4_207_6 : BOOL ;
   Spare_4_207_7 : BOOL ;
   Spare_4_208_0 : BOOL ;
   Spare_4_208_1 : BOOL ;
   Spare_4_208_2 : BOOL ;
   Spare_4_208_3 : BOOL ;
   Spare_4_208_4 : BOOL ;
   Spare_4_208_5 : BOOL ;
   Spare_4_208_6 : BOOL ;
   Spare_4_208_7 : BOOL ;
   Spare_4_209_0 : BOOL ;
   Spare_4_209_1 : BOOL ;
   Spare_4_209_2 : BOOL ;
   Spare_4_209_3 : BOOL ;
   Spare_4_209_4 : BOOL ;
   Spare_4_209_5 : BOOL ;
   Spare_4_209_6 : BOOL ;
   Spare_4_209_7 : BOOL ;
   Spare_4_210 : INT ;
   Spare_4_212 : INT ;
   Spare_4_214 : INT ;
   Spare_4_216 : INT ;
   Spare_4_218 : INT ;
   Spare_4_220 : INT ;
   Spare_4_222 : INT ;
   Spare_4_224 : INT ;
   Spare_4_226 : INT ;
   Spare_4_228 : INT ;
   Spare_4_230 : INT ;
   Spare_4_232 : INT ;
   Spare_4_234 : INT ;	//Block 8 End (32 Bytes)
   PacketNo4B : BYTE ;	//Block 9 (2 Bytes)
   TelegramNo4B : BYTE ;	//Block 9 End (2 Bytes)
   PacketNo5 : BYTE ;	// *** TELEGRAM 5 ***  Block 1 (4 Bytes)
   TelegramNo5 : BYTE ;
   TelegramLength5 : WORD ;	//Block 1 End (4 Bytes)
   DG_9_ENG_COOL_LVL : BOOL ;	//Block 2 (64 Bytes)
   DG_9_ENG_LO_PRESS : BOOL ;
   DG_9_FO_FLT_DIFF_PR : BOOL ;
   DG_9_LO_FLT_DIFF_PR : BOOL ;
   DG_9_ENG_CRK_CASE_PR : BOOL ;
   DG_9_MAR_GEAR_OIL_PR : BOOL ;
   DG_9_ENG_JACK_WT_TEMP_HI : BOOL ;
   DG_9_ENG_JACK_WT_TEMP_LO : BOOL ;
   DG_9_ENG_EXH_GAS_TEMP : BOOL ;
   DG_9_ENG_AFT_COOL_TEMP : BOOL ;
   DG_9_MAR_GEAR_OIL_TEMP : BOOL ;
   DG_9_ENG_OVERSPEED : BOOL ;
   DG_9_EL_FUEL_INJ : BOOL ;
   DG_9_ENG_AIR_RESTR : BOOL ;
   DG_9_SYMMETRIZATION : BOOL ;
   Spare_5_5_7 : BOOL ;
   Spare_5_6_0 : BOOL ;
   Spare_5_6_1 : BOOL ;
   Spare_5_6_2 : BOOL ;
   Spare_5_6_3 : BOOL ;
   Spare_5_6_4 : BOOL ;
   Spare_5_6_5 : BOOL ;
   Spare_5_6_6 : BOOL ;
   Spare_5_6_7 : BOOL ;
   Spare_5_7_0 : BOOL ;
   Spare_5_7_1 : BOOL ;
   Spare_5_7_2 : BOOL ;
   Spare_5_7_3 : BOOL ;
   Spare_5_7_4 : BOOL ;
   Spare_5_7_5 : BOOL ;
   Spare_5_7_6 : BOOL ;
   Spare_5_7_7 : BOOL ;
   Spare_5_8 : INT ;
   Spare_5_10 : INT ;
   Spare_5_12 : INT ;
   Spare_5_14 : INT ;
   Spare_5_16 : INT ;
   Spare_5_18 : INT ;
   Spare_5_20 : INT ;
   Spare_5_22 : INT ;
   Spare_5_24 : INT ;
   Spare_5_26 : INT ;
   Spare_5_28 : INT ;
   Spare_5_30 : INT ;
   DG_9_EXH_GAS_CYL_01_TEMP : INT ;
   DG_9_EXH_GAS_CYL_02_TEMP : INT ;
   DG_9_EXH_GAS_CYL_03_TEMP : INT ;
   DG_9_EXH_GAS_CYL_04_TEMP : INT ;
   DG_9_EXH_GAS_CYL_05_TEMP : INT ;
   DG_9_EXH_GAS_CYL_06_TEMP : INT ;
   DG_9_EXH_GAS_CYL_07_TEMP : INT ;
   DG_9_EXH_GAS_CYL_08_TEMP : INT ;
   DG_9_EXH_GAS_CYL_09_TEMP : INT ;
   DG_9_EXH_GAS_CYL_10_TEMP : INT ;
   DG_9_EXH_GAS_CYL_11_TEMP : INT ;
   DG_9_EXH_GAS_CYL_12_TEMP : INT ;
   DG_9_EXH_GAS_CYL_13_TEMP : INT ;
   DG_9_EXH_GAS_CYL_14_TEMP : INT ;
   DG_9_EXH_GAS_CYL_15_TEMP : INT ;
   DG_9_EXH_GAS_CYL_16_TEMP : INT ;
   DG_9_EXH_CYL_TEMP_MEAN : INT ;
   DG_9_EXH_GAS_TEMP_COMP : INT ;	//Block 2 End (64 Bytes)
   Spare_5_68_0 : BOOL ;
   Spare_5_68_1 : BOOL ;
   Spare_5_68_2 : BOOL ;
   Spare_5_68_3 : BOOL ;
   Spare_5_68_4 : BOOL ;
   Spare_5_68_5 : BOOL ;
   Spare_5_68_6 : BOOL ;
   Spare_5_68_7 : BOOL ;
   Spare_5_69_0 : BOOL ;
   Spare_5_69_1 : BOOL ;
   Spare_5_69_2 : BOOL ;
   Spare_5_69_3 : BOOL ;
   Spare_5_69_4 : BOOL ;
   Spare_5_69_5 : BOOL ;
   Spare_5_69_6 : BOOL ;
   Spare_5_69_7 : BOOL ;
   Spare_5_70_0 : BOOL ;
   Spare_5_70_1 : BOOL ;
   Spare_5_70_2 : BOOL ;
   Spare_5_70_3 : BOOL ;
   Spare_5_70_4 : BOOL ;
   Spare_5_70_5 : BOOL ;
   Spare_5_70_6 : BOOL ;
   Spare_5_70_7 : BOOL ;
   Spare_5_71_0 : BOOL ;
   Spare_5_71_1 : BOOL ;
   Spare_5_71_2 : BOOL ;
   Spare_5_71_3 : BOOL ;
   Spare_5_71_4 : BOOL ;
   Spare_5_71_5 : BOOL ;
   Spare_5_71_6 : BOOL ;
   Spare_5_71_7 : BOOL ;
   Spare_5_72 : INT ;
   Spare_5_74 : INT ;
   Spare_5_76 : INT ;
   Spare_5_78 : INT ;
   Spare_5_80 : INT ;
   Spare_5_82 : INT ;
   Spare_5_84 : INT ;
   Spare_5_86 : INT ;
   Spare_5_88 : INT ;
   Spare_5_90 : INT ;
   Spare_5_92 : INT ;
   Spare_5_94 : INT ;
   Spare_5_96 : INT ;
   Spare_5_98 : INT ;
   Spare_5_100 : INT ;
   Spare_5_102 : INT ;
   Spare_5_104 : INT ;
   Spare_5_106 : INT ;
   Spare_5_108 : INT ;
   Spare_5_110 : INT ;
   Spare_5_112 : INT ;
   Spare_5_114 : INT ;
   Spare_5_116 : INT ;
   Spare_5_118 : INT ;
   Spare_5_120 : INT ;
   Spare_5_122 : INT ;
   Spare_5_124 : INT ;
   Spare_5_126 : INT ;
   Spare_5_128 : INT ;
   Spare_5_130 : INT ;
   GEN_9_VOLTAGE_L1_L2 : INT ;	//Block 4 (32 Bytes)
   GEN_9_VOLTAGE_L1_L3 : INT ;
   GEN_9_VOLTAGE_L2_L3 : INT ;
   GEN_9_CURRENT_L1_L2 : INT ;
   GEN_9_CURRENT_L1_L3 : INT ;
   GEN_9_CURRENT_L2_L3 : INT ;
   GEN_9_ACTIVE_POWER : INT ;
   GEN_9_POWER_FACTOR : INT ;
   GEN_9_REACTIVE_POWER : INT ;
   GEN_9_WDG_TEMP_L1 : INT ;
   GEN_9_WDG_TEMP_L2 : INT ;
   GEN_9_WDG_TEMP_L3 : INT ;
   GEN_9_BEAR_TEMP_DRIVEEND : INT ;
   GEN_9_BEAR_TEMP_NONDRIVE : INT ;
   GEN_9_COOL_AIR_TEMP : INT ;
   GEN_9_COOL_WATER_TEMP : INT ;	//Block_4_End_(32_Bytes)
   GEN_9_MCB_STATUS : BOOL ;	//Block_5_(4_Bytes)
   GEN_9_MCB_SEC_TO_GND : BOOL ;
   GEN_9_Spare : BOOL ;
   GEN_9_OVER_CURRENT_TRIP : BOOL ;
   GEN_9_REVERSE_POWER_TRIP : BOOL ;
   GEN_9_SHORT_CIRCUIT_TRIP : BOOL ;
   GEN_9_Spare2 : BOOL ;
   GEN_9_DIFF_PROT_TRIP : BOOL ;
   Spare_5_165_0 : BOOL ;
   GEN_9_PREFERENTIAL_TRIP : BOOL ;
   GEN_9_BREAKER_TRIP : BOOL ;
   Spare_5_165_3 : BOOL ;
   GEN_9_PMA_71_FAULT : BOOL ;
   GEN_9_W_LEAK_AIR_COOL : BOOL ;
   Spare_5_165_6 : BOOL ;
   Spare_5_165_7 : BOOL ;
   GEN_9_PMA_71_STATUS : WORD ;	//Block 5 End (4 Bytes)
   Spare_5_168 : INT ;	//Block 6 (32 Bytes)
   Spare_5_170 : INT ;
   Spare_5_172 : INT ;
   Spare_5_174 : INT ;
   Spare_5_176 : INT ;
   Spare_5_178 : INT ;
   Spare_5_180 : INT ;
   Spare_5_182 : INT ;
   Spare_5_184 : INT ;
   Spare_5_186 : INT ;
   Spare_5_188 : INT ;
   Spare_5_190 : INT ;
   Spare_5_192 : INT ;
   Spare_5_194 : INT ;
   Spare_5_196 : INT ;
   Spare_5_198 : INT ;	//Block 6 (32 Bytes)
   Spare_5_200_0 : BOOL ;
   Spare_5_200_1 : BOOL ;
   Spare_5_200_2 : BOOL ;
   Spare_5_200_3 : BOOL ;
   Spare_5_200_4 : BOOL ;
   Spare_5_200_5 : BOOL ;
   Spare_5_200_6 : BOOL ;
   Spare_5_200_7 : BOOL ;
   Spare_5_201_0 : BOOL ;
   Spare_5_201_1 : BOOL ;
   Spare_5_201_2 : BOOL ;
   Spare_5_201_3 : BOOL ;
   Spare_5_201_4 : BOOL ;
   Spare_5_201_5 : BOOL ;
   Spare_5_201_6 : BOOL ;
   Spare_5_201_7 : BOOL ;
   Spare_5_202 : WORD ;	//Block 7 End (4 Bytes)
   Spare_5_204_0 : BOOL ;	//Block 8 (32 Bytes)
   Spare_5_204_1 : BOOL ;
   Spare_5_204_2 : BOOL ;
   Spare_5_204_3 : BOOL ;
   Spare_5_204_4 : BOOL ;
   Spare_5_204_5 : BOOL ;
   Spare_5_204_6 : BOOL ;
   Spare_5_204_7 : BOOL ;
   Spare_5_205_0 : BOOL ;
   Spare_5_205_1 : BOOL ;
   Spare_5_205_2 : BOOL ;
   Spare_5_205_3 : BOOL ;
   Spare_5_205_4 : BOOL ;
   Spare_5_205_5 : BOOL ;
   Spare_5_205_6 : BOOL ;
   Spare_5_205_7 : BOOL ;
   Spare_5_206_0 : BOOL ;
   Spare_5_206_1 : BOOL ;
   Spare_5_206_2 : BOOL ;
   Spare_5_206_3 : BOOL ;
   Spare_5_206_4 : BOOL ;
   Spare_5_206_5 : BOOL ;
   Spare_5_206_6 : BOOL ;
   Spare_5_206_7 : BOOL ;
   Spare_5_207_0 : BOOL ;
   Spare_5_207_1 : BOOL ;
   Spare_5_207_2 : BOOL ;
   Spare_5_207_3 : BOOL ;
   Spare_5_207_4 : BOOL ;
   Spare_5_207_5 : BOOL ;
   Spare_5_207_6 : BOOL ;
   Spare_5_207_7 : BOOL ;
   Spare_5_208_0 : BOOL ;
   Spare_5_208_1 : BOOL ;
   Spare_5_208_2 : BOOL ;
   Spare_5_208_3 : BOOL ;
   Spare_5_208_4 : BOOL ;
   Spare_5_208_5 : BOOL ;
   Spare_5_208_6 : BOOL ;
   Spare_5_208_7 : BOOL ;
   Spare_5_209_0 : BOOL ;
   Spare_5_209_1 : BOOL ;
   Spare_5_209_2 : BOOL ;
   Spare_5_209_3 : BOOL ;
   Spare_5_209_4 : BOOL ;
   Spare_5_209_5 : BOOL ;
   Spare_5_209_6 : BOOL ;
   Spare_5_209_7 : BOOL ;
   Spare_5_210 : INT ;
   Spare_5_212 : INT ;
   Spare_5_214 : INT ;
   Spare_5_216 : INT ;
   Spare_5_218 : INT ;
   Spare_5_220 : INT ;
   Spare_5_222 : INT ;
   Spare_5_224 : INT ;
   Spare_5_226 : INT ;
   Spare_5_228 : INT ;
   Spare_5_230 : INT ;
   Spare_5_232 : INT ;
   Spare_5_234 : INT ;	//Block 8 End (32 Bytes)
   PacketNo5B : BYTE ;	//Block 9 (2 Bytes)
   TelegramNo5B : BYTE ;	//Block 9 End (2 Bytes)
  END_STRUCT ;
BEGIN
   PacketNo1 := B#16#0;
   TelegramNo1 := B#16#0;
   TelegramLength1 := W#16#0;
   DG_1_OVERSPEED_TRIP := FALSE;
   DG_1_FUEL_OIL_PRESSURE := FALSE;
   DG_1_INJ_FO_PIPE_LEAK_A := FALSE;
   DG_1_INJ_FO_PIPE_LEAK_B := FALSE;
   DG_1_LUBE_OIL_LEVEL := FALSE;
   DG_1_LO_FLT_DIFF_PR := FALSE;
   DG_1_FO_FLT_DIFF_PR := FALSE;
   Spare_1_4_7 := FALSE;
   DG_1_RUNNING := FALSE;
   DG_1_START_AIR_PRESSURE := FALSE;
   DG_1_SYMMETRIZATION := FALSE;
   Spare_1_5_3 := FALSE;
   Spare_1_5_4 := FALSE;
   Spare_1_5_5 := FALSE;
   Spare_1_5_6 := FALSE;
   Spare_1_5_7 := FALSE;
   Spare_1_6_0 := FALSE;
   Spare_1_6_1 := FALSE;
   Spare_1_6_2 := FALSE;
   Spare_1_6_3 := FALSE;
   Spare_1_6_4 := FALSE;
   Spare_1_6_5 := FALSE;
   Spare_1_6_6 := FALSE;
   Spare_1_6_7 := FALSE;
   Spare_1_7_0 := FALSE;
   Spare_1_7_1 := FALSE;
   Spare_1_7_2 := FALSE;
   Spare_1_7_3 := FALSE;
   Spare_1_7_4 := FALSE;
   Spare_1_7_5 := FALSE;
   Spare_1_7_6 := FALSE;
   Spare_1_7_7 := FALSE;
   DG_1_LO_PRESSURE := 0;
   DG_1_FUEL_OIL_PRESSUREA := 0;
   DG_1_HT_CW_PRESSURE := 0;
   DG_1_CA_PRESSURE := 0;
   DG_1_INJ_COOL_OIL_PRESS := 0;
   DG_1_RPM := 0;
   DG_1_TURBO_CHARGER_A_RPM := 0;
   DG_1_TURBO_CHARGER_B_RPM := 0;
   DG_1_LO_TEMP := 0;
   DG_1_COOL_WATER_TEMP := 0;
   DG_1_CHARG_AIR_TEMP := 0;
   DG_1_INJ_COOL_OIL_TEMP := 0;
   DG_1_EXH_GAS_CYL_01_TEMP := 0;
   DG_1_EXH_GAS_CYL_02_TEMP := 0;
   DG_1_EXH_GAS_CYL_03_TEMP := 0;
   DG_1_EXH_GAS_CYL_04_TEMP := 0;
   DG_1_EXH_GAS_CYL_05_TEMP := 0;
   DG_1_EXH_GAS_CYL_06_TEMP := 0;
   DG_1_EXH_GAS_CYL_07_TEMP := 0;
   DG_1_EXH_GAS_CYL_08_TEMP := 0;
   DG_1_EXH_GAS_CYL_09_TEMP := 0;
   DG_1_EXH_GAS_CYL_10_TEMP := 0;
   DG_1_EXH_GAS_CYL_11_TEMP := 0;
   DG_1_EXH_GAS_CYL_12_TEMP := 0;
   DG_1_EXH_GAS_CYL_13_TEMP := 0;
   DG_1_EXH_GAS_CYL_14_TEMP := 0;
   DG_1_EXH_GAS_CYL_15_TEMP := 0;
   DG_1_EXH_GAS_CYL_16_TEMP := 0;
   DG_1_EXH_CYL_TEMP_MEAN := 0;
   DG_1_EXH_GAS_TEMP_COMP := 0;
   DG_2_OVERSPEED_TRIP := FALSE;
   DG_2_FUEL_OIL_PRES := FALSE;
   DG_2_INJ_FO_PIPE_LEAK_A := FALSE;
   DG_2_INJ_FO_PIPE_LEAK_B := FALSE;
   DG_2_ENGINE_LUBE_OIL_LVL := FALSE;
   DG_2_LO_FLT_DIFF_PR := FALSE;
   DG_2_FO_FLT_DIFF_PR := FALSE;
   Spare_1_68_7 := FALSE;
   DG_2_ENGINE_RUNNING := FALSE;
   DG_2_START_AIR_PRESSURE := FALSE;
   DG_2_SYMMETRIZATION := FALSE;
   Spare_1_69_3 := FALSE;
   Spare_1_69_4 := FALSE;
   Spare_1_69_5 := FALSE;
   Spare_1_69_6 := FALSE;
   Spare_1_69_7 := FALSE;
   Spare_1_70_0 := FALSE;
   Spare_1_70_1 := FALSE;
   Spare_1_70_2 := FALSE;
   Spare_1_70_3 := FALSE;
   Spare_1_70_4 := FALSE;
   Spare_1_70_5 := FALSE;
   Spare_1_70_6 := FALSE;
   Spare_1_70_7 := FALSE;
   Spare_1_71_0 := FALSE;
   Spare_1_71_1 := FALSE;
   Spare_1_71_2 := FALSE;
   Spare_1_71_3 := FALSE;
   Spare_1_71_4 := FALSE;
   Spare_1_71_5 := FALSE;
   Spare_1_71_6 := FALSE;
   Spare_1_71_7 := FALSE;
   DG_2_ENGINE_LO_PRESSURE := 0;
   DG_2_FUEL_OIL_PRESA := 0;
   DG_2_HT_CW_PRESSURE := 0;
   DG_2_CA_PRESSURE := 0;
   DG_2_INJ_COOL_OIL_PRESS := 0;
   DG_2_ENGINE_RPM := 0;
   DG_2_TURBO_CHARGER_A_RPM := 0;
   DG_2_TURBO_CHARGER_B_RPM := 0;
   DG_2_ENGINE_LO_TEMP := 0;
   DG_2_COOL_WATER_TEMP := 0;
   DG_2_CHARG_AIR_TEMP := 0;
   DG_2_INJ_COOL_OIL_TEMP := 0;
   DG_2_EXH_GAS_CYL_01_TEMP := 0;
   DG_2_EXH_GAS_CYL_02_TEMP := 0;
   DG_2_EXH_GAS_CYL_03_TEMP := 0;
   DG_2_EXH_GAS_CYL_04_TEMP := 0;
   DG_2_EXH_GAS_CYL_05_TEMP := 0;
   DG_2_EXH_GAS_CYL_06_TEMP := 0;
   DG_2_EXH_GAS_CYL_07_TEMP := 0;
   DG_2_EXH_GAS_CYL_08_TEMP := 0;
   DG_2_EXH_GAS_CYL_09_TEMP := 0;
   DG_2_EXH_GAS_CYL_10_TEMP := 0;
   DG_2_EXH_GAS_CYL_11_TEMP := 0;
   DG_2_EXH_GAS_CYL_12_TEMP := 0;
   DG_2_EXH_GAS_CYL_13_TEMP := 0;
   DG_2_EXH_GAS_CYL_14_TEMP := 0;
   DG_2_EXH_GAS_CYL_15_TEMP := 0;
   DG_2_EXH_GAS_CYL_16_TEMP := 0;
   DG_2_EXH_CYL_TEMP_MEAN := 0;
   DG_2_EXH_GAS_TEMP_COMP := 0;
   GEN_1_VOLTAGE_L1_L2 := 0;
   GEN_1_VOLTAGE_L1_L3 := 0;
   GEN_1_VOLTAGE_L2_L3 := 0;
   GEN_1_CURRENT_L1_L2 := 0;
   GEN_1_CURRENT_L1_L3 := 0;
   GEN_1_CURRENT_L2_L3 := 0;
   GEN_1_ACTIVE_POWER := 0;
   GEN_1_POWER_FACTOR := 0;
   GEN_1_REACTIVE_POWER := 0;
   GEN_1_WDG_TEMP_L1 := 0;
   GEN_1_WDG_TEMP_L2 := 0;
   GEN_1_WDG_TEMP_L3 := 0;
   GEN_1_BEAR_TEMP_DRIVEEND := 0;
   GEN_1_BEAR_TEMP_NONDRIVE := 0;
   GEN_1_COOL_AIR_TEMP := 0;
   GEN_1_COOL_WATER_TEMP := 0;
   GEN_1_MCB_STATUS := FALSE;
   GEN_1_MCB_SEC_TO_GND := FALSE;
   GEN_1_Spare := FALSE;
   GEN_1_OVER_CURRENT_TRIP := FALSE;
   GEN_1_REVERSE_POWER_TRIP := FALSE;
   GEN_1_SHORT_CIRCUIT_TRIP := FALSE;
   GEN_1_Spare2 := FALSE;
   GEN_1_DIFF_PROT_TRIP := FALSE;
   Spare_1_165_0 := FALSE;
   GEN_1_PREFERENTIAL_TRIP := FALSE;
   GEN_1_BREAKER_TRIP := FALSE;
   Spare_1_165_3 := FALSE;
   GEN_1_PMA_71_FAULT := FALSE;
   GEN_1_W_LEAK_AIR_COOL := FALSE;
   Spare_1_165_6 := FALSE;
   Spare_1_165_7 := FALSE;
   GEN_1_PMA_71_STATUS := W#16#0;
   GEN_2_VOLTAGE_L1_L2 := 0;
   GEN_2_VOLTAGE_L1_L3 := 0;
   GEN_2_VOLTAGE_L2_L3 := 0;
   GEN_2_CURRENT_L1_L2 := 0;
   GEN_2_CURRENT_L1_L3 := 0;
   GEN_2_CURRENT_L2_L3 := 0;
   GEN_2_ACTIVE_POWER := 0;
   GEN_2_POWER_FACTOR := 0;
   GEN_2_REACTIVE_POWER := 0;
   GEN_2_WDG_TEMP_L1 := 0;
   GEN_2_WDG_TEMP_L2 := 0;
   GEN_2_WDG_TEMP_L3 := 0;
   GEN_2_BEAR_TEMP_DRIVEEND := 0;
   GEN_2_BEAR_TEMP_NONDRIVE := 0;
   GEN_2_COOL_AIR_TEMP := 0;
   GEN_2_COOL_WATER_TEMP := 0;
   GEN_2_MCB_STATUS := FALSE;
   GEN_2_MCB_SEC_TO_GND := FALSE;
   GEN_2_Spare := FALSE;
   GEN_2_OVER_CURRENT_TRIP := FALSE;
   GEN_2_REVERSE_POWER_TRIP := FALSE;
   GEN_2_SHORT_CIRCUIT_TRIP := FALSE;
   GEN_2_Spare2 := FALSE;
   GEN_2_DIFF_PROT_TRIP := FALSE;
   Spare_1_201_0 := FALSE;
   GEN_2_PREFERENTIAL_TRIP := FALSE;
   GEN_2_BREAKER_TRIP := FALSE;
   Spare_1_201_3 := FALSE;
   GEN_2_PMA_71_FAULT := FALSE;
   GEN_2_W_LEAK_AIR_COOL := FALSE;
   Spare_1_201_6 := FALSE;
   Spare_1_201_7 := FALSE;
   GEN_2_PMA_71_STATUS := W#16#0;
   Spare_1_204_0 := FALSE;
   Spare_1_204_1 := FALSE;
   Spare_1_204_2 := FALSE;
   Spare_1_204_3 := FALSE;
   Spare_1_204_4 := FALSE;
   Spare_1_204_5 := FALSE;
   Spare_1_204_6 := FALSE;
   Spare_1_204_7 := FALSE;
   Spare_1_205_0 := FALSE;
   Spare_1_205_1 := FALSE;
   Spare_1_205_2 := FALSE;
   Spare_1_205_3 := FALSE;
   Spare_1_205_4 := FALSE;
   Spare_1_205_5 := FALSE;
   Spare_1_205_6 := FALSE;
   Spare_1_205_7 := FALSE;
   Spare_1_206_0 := FALSE;
   Spare_1_206_1 := FALSE;
   Spare_1_206_2 := FALSE;
   Spare_1_206_3 := FALSE;
   Spare_1_206_4 := FALSE;
   Spare_1_206_5 := FALSE;
   Spare_1_206_6 := FALSE;
   Spare_1_206_7 := FALSE;
   Spare_1_207_0 := FALSE;
   Spare_1_207_1 := FALSE;
   Spare_1_207_2 := FALSE;
   Spare_1_207_3 := FALSE;
   Spare_1_207_4 := FALSE;
   Spare_1_207_5 := FALSE;
   Spare_1_207_6 := FALSE;
   Spare_1_207_7 := FALSE;
   Spare_1_208_0 := FALSE;
   Spare_1_208_1 := FALSE;
   Spare_1_208_2 := FALSE;
   Spare_1_208_3 := FALSE;
   Spare_1_208_4 := FALSE;
   Spare_1_208_5 := FALSE;
   Spare_1_208_6 := FALSE;
   Spare_1_208_7 := FALSE;
   Spare_1_209_0 := FALSE;
   Spare_1_209_1 := FALSE;
   Spare_1_209_2 := FALSE;
   Spare_1_209_3 := FALSE;
   Spare_1_209_4 := FALSE;
   Spare_1_209_5 := FALSE;
   Spare_1_209_6 := FALSE;
   Spare_1_209_7 := FALSE;
   LV_TRANSF_1_WDG_L1_TEMP := 0;
   LV_TRANSF_1_WDG_L2_TEMP := 0;
   LV_TRANSF_1_WDG_L3_TEMP := 0;
   LV_TRANSF_2_WDG_L1_TEMP := 0;
   LV_TRANSF_2_WDG_L2_TEMP := 0;
   LV_TRANSF_2_WDG_L3_TEMP := 0;
   STRT_AIR_PRESS_BOTTLE_1 := 0;
   STRT_AIR_PRESS_BOTTLE_2 := 0;
   STRT_AIR_BOT_CAT_PRESS := 0;
   Spare_1_228 := 0;
   Spare_1_230 := 0;
   Spare_1_232 := 0;
   Spare_1_234 := 0;
   PacketNo1B := B#16#0;
   TelegramNo1B := B#16#0;
   PacketNo2 := B#16#0;
   TelegramNo2 := B#16#0;
   TelegramLength2 := W#16#0;
   DG_3_OVERSPEED_TRIP := FALSE;
   DG_3_FUEL_OIL_PRESSURE := FALSE;
   DG_3_INJ_FO_PIPE_LEAK_A := FALSE;
   DG_3_INJ_FO_PIPE_LEAK_B := FALSE;
   DG_3_LUBE_OIL_LEVEL := FALSE;
   DG_3_LO_FLT_DIFF_PR := FALSE;
   DG_3_FO_FLT_DIFF_PR := FALSE;
   Spare_2_4_7 := FALSE;
   DG_3_RUNNING := FALSE;
   DG_3_START_AIR_PRESSURE := FALSE;
   DG_3_SYMMETRIZATION := FALSE;
   Spare_2_5_3 := FALSE;
   Spare_2_5_4 := FALSE;
   Spare_2_5_5 := FALSE;
   Spare_2_5_6 := FALSE;
   Spare_2_5_7 := FALSE;
   Spare_2_6_0 := FALSE;
   Spare_2_6_1 := FALSE;
   Spare_2_6_2 := FALSE;
   Spare_2_6_3 := FALSE;
   Spare_2_6_4 := FALSE;
   Spare_2_6_5 := FALSE;
   Spare_2_6_6 := FALSE;
   Spare_2_6_7 := FALSE;
   Spare_2_7_0 := FALSE;
   Spare_2_7_1 := FALSE;
   Spare_2_7_2 := FALSE;
   Spare_2_7_3 := FALSE;
   Spare_2_7_4 := FALSE;
   Spare_2_7_5 := FALSE;
   Spare_2_7_6 := FALSE;
   Spare_2_7_7 := FALSE;
   DG_3_LO_PRESSURE := 0;
   DG_3_FUEL_OIL_PRESSUREA := 0;
   DG_3_HT_CW_PRESSURE := 0;
   DG_3_CA_PRESSURE := 0;
   DG_3_INJ_COOL_OIL_PRESS := 0;
   DG_3_RPM := 0;
   DG_3_TURBO_CHARGER_A_RPM := 0;
   DG_3_TURBO_CHARGER_B_RPM := 0;
   DG_3_LO_TEMP := 0;
   DG_3_COOL_WATER_TEMP := 0;
   DG_3_CHARG_AIR_TEMP := 0;
   DG_3_INJ_COOL_OIL_TEMP := 0;
   DG_3_EXH_GAS_CYL_01_TEMP := 0;
   DG_3_EXH_GAS_CYL_02_TEMP := 0;
   DG_3_EXH_GAS_CYL_03_TEMP := 0;
   DG_3_EXH_GAS_CYL_04_TEMP := 0;
   DG_3_EXH_GAS_CYL_05_TEMP := 0;
   DG_3_EXH_GAS_CYL_06_TEMP := 0;
   DG_3_EXH_GAS_CYL_07_TEMP := 0;
   DG_3_EXH_GAS_CYL_08_TEMP := 0;
   DG_3_EXH_GAS_CYL_09_TEMP := 0;
   DG_3_EXH_GAS_CYL_10_TEMP := 0;
   DG_3_EXH_GAS_CYL_11_TEMP := 0;
   DG_3_EXH_GAS_CYL_12_TEMP := 0;
   DG_3_EXH_GAS_CYL_13_TEMP := 0;
   DG_3_EXH_GAS_CYL_14_TEMP := 0;
   DG_3_EXH_GAS_CYL_15_TEMP := 0;
   DG_3_EXH_GAS_CYL_16_TEMP := 0;
   DG_3_EXH_CYL_TEMP_MEAN := 0;
   DG_3_EXH_GAS_TEMP_COMP := 0;
   DG_4_OVERSPEED_TRIP := FALSE;
   DG_4_FUEL_OIL_PRES := FALSE;
   DG_4_INJ_FO_PIPE_LEAK_A := FALSE;
   DG_4_INJ_FO_PIPE_LEAK_B := FALSE;
   DG_4_ENGINE_LUBE_OIL_LVL := FALSE;
   DG_4_LO_FLT_DIFF_PR := FALSE;
   DG_4_FO_FLT_DIFF_PR := FALSE;
   Spare_2_68_7 := FALSE;
   DG_4_ENGINE_RUNNING := FALSE;
   DG_4_START_AIR_PRESSURE := FALSE;
   DG_4_SYMMETRIZATION := FALSE;
   Spare_2_69_3 := FALSE;
   Spare_2_69_4 := FALSE;
   Spare_2_69_5 := FALSE;
   Spare_2_69_6 := FALSE;
   Spare_2_69_7 := FALSE;
   Spare_2_70_0 := FALSE;
   Spare_2_70_1 := FALSE;
   Spare_2_70_2 := FALSE;
   Spare_2_70_3 := FALSE;
   Spare_2_70_4 := FALSE;
   Spare_2_70_5 := FALSE;
   Spare_2_70_6 := FALSE;
   Spare_2_70_7 := FALSE;
   Spare_2_71_0 := FALSE;
   Spare_2_71_1 := FALSE;
   Spare_2_71_2 := FALSE;
   Spare_2_71_3 := FALSE;
   Spare_2_71_4 := FALSE;
   Spare_2_71_5 := FALSE;
   Spare_2_71_6 := FALSE;
   Spare_2_71_7 := FALSE;
   DG_4_ENGINE_LO_PRESSURE := 0;
   DG_4_FUEL_OIL_PRESA := 0;
   DG_4_HT_CW_PRESSURE := 0;
   DG_4_CA_PRESSURE := 0;
   DG_4_INJ_COOL_OIL_PRESS := 0;
   DG_4_ENGINE_RPM := 0;
   DG_4_TURBO_CHARGER_A_RPM := 0;
   DG_4_TURBO_CHARGER_B_RPM := 0;
   DG_4_ENGINE_LO_TEMP := 0;
   DG_4_COOL_WATER_TEMP := 0;
   DG_4_CHARG_AIR_TEMP := 0;
   DG_4_INJ_COOL_OIL_TEMP := 0;
   DG_4_EXH_GAS_CYL_01_TEMP := 0;
   DG_4_EXH_GAS_CYL_02_TEMP := 0;
   DG_4_EXH_GAS_CYL_03_TEMP := 0;
   DG_4_EXH_GAS_CYL_04_TEMP := 0;
   DG_4_EXH_GAS_CYL_05_TEMP := 0;
   DG_4_EXH_GAS_CYL_06_TEMP := 0;
   DG_4_EXH_GAS_CYL_07_TEMP := 0;
   DG_4_EXH_GAS_CYL_08_TEMP := 0;
   DG_4_EXH_GAS_CYL_09_TEMP := 0;
   DG_4_EXH_GAS_CYL_10_TEMP := 0;
   DG_4_EXH_GAS_CYL_11_TEMP := 0;
   DG_4_EXH_GAS_CYL_12_TEMP := 0;
   DG_4_EXH_GAS_CYL_13_TEMP := 0;
   DG_4_EXH_GAS_CYL_14_TEMP := 0;
   DG_4_EXH_GAS_CYL_15_TEMP := 0;
   DG_4_EXH_GAS_CYL_16_TEMP := 0;
   DG_4_EXH_CYL_TEMP_MEAN := 0;
   DG_4_EXH_GAS_TEMP_COMP := 0;
   GEN_3_VOLTAGE_L1_L2 := 0;
   GEN_3_VOLTAGE_L1_L3 := 0;
   GEN_3_VOLTAGE_L2_L3 := 0;
   GEN_3_CURRENT_L1_L2 := 0;
   GEN_3_CURRENT_L1_L3 := 0;
   GEN_3_CURRENT_L2_L3 := 0;
   GEN_3_ACTIVE_POWER := 0;
   GEN_3_POWER_FACTOR := 0;
   GEN_3_REACTIVE_POWER := 0;
   GEN_3_WDG_TEMP_L1 := 0;
   GEN_3_WDG_TEMP_L2 := 0;
   GEN_3_WDG_TEMP_L3 := 0;
   GEN_3_BEAR_TEMP_DRIVEEND := 0;
   GEN_3_BEAR_TEMP_NONDRIVE := 0;
   GEN_3_COOL_AIR_TEMP := 0;
   GEN_3_COOL_WATER_TEMP := 0;
   GEN_3_MCB_STATUS := FALSE;
   GEN_3_MCB_SEC_TO_GND := FALSE;
   GEN_3_Spare := FALSE;
   GEN_3_OVER_CURRENT_TRIP := FALSE;
   GEN_3_REVERSE_POWER_TRIP := FALSE;
   GEN_3_SHORT_CIRCUIT_TRIP := FALSE;
   GEN_3_Spare2 := FALSE;
   GEN_3_DIFF_PROT_TRIP := FALSE;
   Spare_2_165_0 := FALSE;
   GEN_3_PREFERENTIAL_TRIP := FALSE;
   GEN_3_BREAKER_TRIP := FALSE;
   Spare_2_165_3 := FALSE;
   GEN_3_PMA_71_FAULT := FALSE;
   GEN_3_W_LEAK_AIR_COOL := FALSE;
   Spare_2_165_6 := FALSE;
   Spare_2_165_7 := FALSE;
   GEN_3_PMA_71_STATUS := W#16#0;
   GEN_4_VOLTAGE_L1_L2 := 0;
   GEN_4_VOLTAGE_L1_L3 := 0;
   GEN_4_VOLTAGE_L2_L3 := 0;
   GEN_4_CURRENT_L1_L2 := 0;
   GEN_4_CURRENT_L1_L3 := 0;
   GEN_4_CURRENT_L2_L3 := 0;
   GEN_4_ACTIVE_POWER := 0;
   GEN_4_POWER_FACTOR := 0;
   GEN_4_REACTIVE_POWER := 0;
   GEN_4_WDG_TEMP_L1 := 0;
   GEN_4_WDG_TEMP_L2 := 0;
   GEN_4_WDG_TEMP_L3 := 0;
   GEN_4_BEAR_TEMP_DRIVEEND := 0;
   GEN_4_BEAR_TEMP_NONDRIVE := 0;
   GEN_4_COOL_AIR_TEMP := 0;
   GEN_4_COOL_WATER_TEMP := 0;
   GEN_4_MCB_STATUS := FALSE;
   GEN_4_MCB_SEC_TO_GND := FALSE;
   GEN_4_Spare := FALSE;
   GEN_4_OVER_CURRENT_TRIP := FALSE;
   GEN_4_REVERSE_POWER_TRIP := FALSE;
   GEN_4_SHORT_CIRCUIT_TRIP := FALSE;
   GEN_4_Spare2 := FALSE;
   GEN_4_DIFF_PROT_TRIP := FALSE;
   Spare_2_201_0 := FALSE;
   GEN_4_PREFERENTIAL_TRIP := FALSE;
   GEN_4_BREAKER_TRIP := FALSE;
   Spare_2_201_3 := FALSE;
   GEN_4_PMA_71_FAULT := FALSE;
   GEN_4_W_LEAK_AIR_COOL := FALSE;
   Spare_2_201_6 := FALSE;
   Spare_2_201_7 := FALSE;
   GEN_4_PMA_71_STATUS := W#16#0;
   Spare_2_204_0 := FALSE;
   Spare_2_204_1 := FALSE;
   Spare_2_204_2 := FALSE;
   Spare_2_204_3 := FALSE;
   Spare_2_204_4 := FALSE;
   Spare_2_204_5 := FALSE;
   Spare_2_204_6 := FALSE;
   Spare_2_204_7 := FALSE;
   Spare_2_205_0 := FALSE;
   Spare_2_205_1 := FALSE;
   Spare_2_205_2 := FALSE;
   Spare_2_205_3 := FALSE;
   Spare_2_205_4 := FALSE;
   Spare_2_205_5 := FALSE;
   Spare_2_205_6 := FALSE;
   Spare_2_205_7 := FALSE;
   Spare_2_206_0 := FALSE;
   Spare_2_206_1 := FALSE;
   Spare_2_206_2 := FALSE;
   Spare_2_206_3 := FALSE;
   Spare_2_206_4 := FALSE;
   Spare_2_206_5 := FALSE;
   Spare_2_206_6 := FALSE;
   Spare_2_206_7 := FALSE;
   Spare_2_207_0 := FALSE;
   Spare_2_207_1 := FALSE;
   Spare_2_207_2 := FALSE;
   Spare_2_207_3 := FALSE;
   Spare_2_207_4 := FALSE;
   Spare_2_207_5 := FALSE;
   Spare_2_207_6 := FALSE;
   Spare_2_207_7 := FALSE;
   Spare_2_208_0 := FALSE;
   Spare_2_208_1 := FALSE;
   Spare_2_208_2 := FALSE;
   Spare_2_208_3 := FALSE;
   Spare_2_208_4 := FALSE;
   Spare_2_208_5 := FALSE;
   Spare_2_208_6 := FALSE;
   Spare_2_208_7 := FALSE;
   Spare_2_209_0 := FALSE;
   Spare_2_209_1 := FALSE;
   Spare_2_209_2 := FALSE;
   Spare_2_209_3 := FALSE;
   Spare_2_209_4 := FALSE;
   Spare_2_209_5 := FALSE;
   Spare_2_209_6 := FALSE;
   Spare_2_209_7 := FALSE;
   Spare_2_210 := 0;
   Spare_2_212 := 0;
   Spare_2_214 := 0;
   Spare_2_216 := 0;
   Spare_2_218 := 0;
   Spare_2_220 := 0;
   Spare_2_222 := 0;
   Spare_2_224 := 0;
   Spare_2_226 := 0;
   Spare_2_228 := 0;
   Spare_2_230 := 0;
   Spare_2_232 := 0;
   Spare_2_234 := 0;
   PacketNo2B := B#16#0;
   TelegramNo2B := B#16#0;
   PacketNo3 := B#16#0;
   TelegramNo3 := B#16#0;
   TelegramLength3 := W#16#0;
   DG_5_OVERSPEED_TRIP := FALSE;
   DG_5_FUEL_OIL_PRESSURE := FALSE;
   DG_5_INJ_FO_PIPE_LEAK_A := FALSE;
   DG_5_INJ_FO_PIPE_LEAK_B := FALSE;
   DG_5_LUBE_OIL_LEVEL := FALSE;
   DG_5_LO_FLT_DIFF_PR := FALSE;
   DG_5_FO_FLT_DIFF_PR := FALSE;
   Spare_3_4_7 := FALSE;
   DG_5_RUNNING := FALSE;
   DG_5_START_AIR_PRESSURE := FALSE;
   DG_5_SYMMETRIZATION := FALSE;
   Spare_3_5_3 := FALSE;
   Spare_3_5_4 := FALSE;
   Spare_3_5_5 := FALSE;
   Spare_3_5_6 := FALSE;
   Spare_3_5_7 := FALSE;
   Spare_3_6_0 := FALSE;
   Spare_3_6_1 := FALSE;
   Spare_3_6_2 := FALSE;
   Spare_3_6_3 := FALSE;
   Spare_3_6_4 := FALSE;
   Spare_3_6_5 := FALSE;
   Spare_3_6_6 := FALSE;
   Spare_3_6_7 := FALSE;
   Spare_3_7_0 := FALSE;
   Spare_3_7_1 := FALSE;
   Spare_3_7_2 := FALSE;
   Spare_3_7_3 := FALSE;
   Spare_3_7_4 := FALSE;
   Spare_3_7_5 := FALSE;
   Spare_3_7_6 := FALSE;
   Spare_3_7_7 := FALSE;
   DG_5_LO_PRESSURE := 0;
   DG_5_FUEL_OIL_PRESSUREA := 0;
   DG_5_HT_CW_PRESSURE := 0;
   DG_5_CA_PRESSURE := 0;
   DG_5_INJ_COOL_OIL_PRESS := 0;
   DG_5_RPM := 0;
   DG_5_TURBO_CHARGER_A_RPM := 0;
   DG_5_TURBO_CHARGER_B_RPM := 0;
   DG_5_LO_TEMP := 0;
   DG_5_COOL_WATER_TEMP := 0;
   DG_5_CHARG_AIR_TEMP := 0;
   DG_5_INJ_COOL_OIL_TEMP := 0;
   DG_5_EXH_GAS_CYL_01_TEMP := 0;
   DG_5_EXH_GAS_CYL_02_TEMP := 0;
   DG_5_EXH_GAS_CYL_03_TEMP := 0;
   DG_5_EXH_GAS_CYL_04_TEMP := 0;
   DG_5_EXH_GAS_CYL_05_TEMP := 0;
   DG_5_EXH_GAS_CYL_06_TEMP := 0;
   DG_5_EXH_GAS_CYL_07_TEMP := 0;
   DG_5_EXH_GAS_CYL_08_TEMP := 0;
   DG_5_EXH_GAS_CYL_09_TEMP := 0;
   DG_5_EXH_GAS_CYL_10_TEMP := 0;
   DG_5_EXH_GAS_CYL_11_TEMP := 0;
   DG_5_EXH_GAS_CYL_12_TEMP := 0;
   DG_5_EXH_GAS_CYL_13_TEMP := 0;
   DG_5_EXH_GAS_CYL_14_TEMP := 0;
   DG_5_EXH_GAS_CYL_15_TEMP := 0;
   DG_5_EXH_GAS_CYL_16_TEMP := 0;
   DG_5_EXH_CYL_TEMP_MEAN := 0;
   DG_5_EXH_GAS_TEMP_COMP := 0;
   DG_6_OVERSPEED_TRIP := FALSE;
   DG_6_FUEL_OIL_PRES := FALSE;
   DG_6_INJ_FO_PIPE_LEAK_A := FALSE;
   DG_6_INJ_FO_PIPE_LEAK_B := FALSE;
   DG_6_ENGINE_LUBE_OIL_LVL := FALSE;
   DG_6_LO_FLT_DIFF_PR := FALSE;
   DG_6_FO_FLT_DIFF_PR := FALSE;
   Spare_3_68_7 := FALSE;
   DG_6_ENGINE_RUNNING := FALSE;
   DG_6_START_AIR_PRESSURE := FALSE;
   DG_6_SYMMETRIZATION := FALSE;
   Spare_3_69_3 := FALSE;
   Spare_3_69_4 := FALSE;
   Spare_3_69_5 := FALSE;
   Spare_3_69_6 := FALSE;
   Spare_3_69_7 := FALSE;
   Spare_3_70_0 := FALSE;
   Spare_3_70_1 := FALSE;
   Spare_3_70_2 := FALSE;
   Spare_3_70_3 := FALSE;
   Spare_3_70_4 := FALSE;
   Spare_3_70_5 := FALSE;
   Spare_3_70_6 := FALSE;
   Spare_3_70_7 := FALSE;
   Spare_3_71_0 := FALSE;
   Spare_3_71_1 := FALSE;
   Spare_3_71_2 := FALSE;
   Spare_3_71_3 := FALSE;
   Spare_3_71_4 := FALSE;
   Spare_3_71_5 := FALSE;
   Spare_3_71_6 := FALSE;
   Spare_3_71_7 := FALSE;
   DG_6_ENGINE_LO_PRESSURE := 0;
   DG_6_FUEL_OIL_PRESA := 0;
   DG_6_HT_CW_PRESSURE := 0;
   DG_6_CA_PRESSURE := 0;
   DG_6_INJ_COOL_OIL_PRESS := 0;
   DG_6_ENGINE_RPM := 0;
   DG_6_TURBO_CHARGER_A_RPM := 0;
   DG_6_TURBO_CHARGER_B_RPM := 0;
   DG_6_ENGINE_LO_TEMP := 0;
   DG_6_COOL_WATER_TEMP := 0;
   DG_6_CHARG_AIR_TEMP := 0;
   DG_6_INJ_COOL_OIL_TEMP := 0;
   DG_6_EXH_GAS_CYL_01_TEMP := 0;
   DG_6_EXH_GAS_CYL_02_TEMP := 0;
   DG_6_EXH_GAS_CYL_03_TEMP := 0;
   DG_6_EXH_GAS_CYL_04_TEMP := 0;
   DG_6_EXH_GAS_CYL_05_TEMP := 0;
   DG_6_EXH_GAS_CYL_06_TEMP := 0;
   DG_6_EXH_GAS_CYL_07_TEMP := 0;
   DG_6_EXH_GAS_CYL_08_TEMP := 0;
   DG_6_EXH_GAS_CYL_09_TEMP := 0;
   DG_6_EXH_GAS_CYL_10_TEMP := 0;
   DG_6_EXH_GAS_CYL_11_TEMP := 0;
   DG_6_EXH_GAS_CYL_12_TEMP := 0;
   DG_6_EXH_GAS_CYL_13_TEMP := 0;
   DG_6_EXH_GAS_CYL_14_TEMP := 0;
   DG_6_EXH_GAS_CYL_15_TEMP := 0;
   DG_6_EXH_GAS_CYL_16_TEMP := 0;
   DG_6_EXH_CYL_TEMP_MEAN := 0;
   DG_6_EXH_GAS_TEMP_COMP := 0;
   GEN_5_VOLTAGE_L1_L2 := 0;
   GEN_5_VOLTAGE_L1_L3 := 0;
   GEN_5_VOLTAGE_L2_L3 := 0;
   GEN_5_CURRENT_L1_L2 := 0;
   GEN_5_CURRENT_L1_L3 := 0;
   GEN_5_CURRENT_L2_L3 := 0;
   GEN_5_ACTIVE_POWER := 0;
   GEN_5_POWER_FACTOR := 0;
   GEN_5_REACTIVE_POWER := 0;
   GEN_5_WDG_TEMP_L1 := 0;
   GEN_5_WDG_TEMP_L2 := 0;
   GEN_5_WDG_TEMP_L3 := 0;
   GEN_5_BEAR_TEMP_DRIVEEND := 0;
   GEN_5_BEAR_TEMP_NONDRIVE := 0;
   GEN_5_COOL_AIR_TEMP := 0;
   GEN_5_COOL_WATER_TEMP := 0;
   GEN_5_MCB_STATUS := FALSE;
   GEN_5_MCB_SEC_TO_GND := FALSE;
   GEN_5_Spare := FALSE;
   GEN_5_OVER_CURRENT_TRIP := FALSE;
   GEN_5_REVERSE_POWER_TRIP := FALSE;
   GEN_5_SHORT_CIRCUIT_TRIP := FALSE;
   GEN_5_Spare2 := FALSE;
   GEN_5_DIFF_PROT_TRIP := FALSE;
   Spare_3_165_0 := FALSE;
   GEN_5_PREFERENTIAL_TRIP := FALSE;
   GEN_5_BREAKER_TRIP := FALSE;
   Spare_3_165_3 := FALSE;
   GEN_5_PMA_71_FAULT := FALSE;
   GEN_5_W_LEAK_AIR_COOL := FALSE;
   Spare_3_165_6 := FALSE;
   Spare_3_165_7 := FALSE;
   GEN_5_PMA_71_STATUS := W#16#0;
   GEN_6_VOLTAGE_L1_L2 := 0;
   GEN_6_VOLTAGE_L1_L3 := 0;
   GEN_6_VOLTAGE_L2_L3 := 0;
   GEN_6_CURRENT_L1_L2 := 0;
   GEN_6_CURRENT_L1_L3 := 0;
   GEN_6_CURRENT_L2_L3 := 0;
   GEN_6_ACTIVE_POWER := 0;
   GEN_6_POWER_FACTOR := 0;
   GEN_6_REACTIVE_POWER := 0;
   GEN_6_WDG_TEMP_L1 := 0;
   GEN_6_WDG_TEMP_L2 := 0;
   GEN_6_WDG_TEMP_L3 := 0;
   GEN_6_BEAR_TEMP_DRIVEEND := 0;
   GEN_6_BEAR_TEMP_NONDRIVE := 0;
   GEN_6_COOL_AIR_TEMP := 0;
   GEN_6_COOL_WATER_TEMP := 0;
   GEN_6_MCB_STATUS := FALSE;
   GEN_6_MCB_SEC_TO_GND := FALSE;
   GEN_6_Spare := FALSE;
   GEN_6_OVER_CURRENT_TRIP := FALSE;
   GEN_6_REVERSE_POWER_TRIP := FALSE;
   GEN_6_SHORT_CIRCUIT_TRIP := FALSE;
   GEN_6_Spare2 := FALSE;
   GEN_6_DIFF_PROT_TRIP := FALSE;
   Spare_3_201_0 := FALSE;
   GEN_6_PREFERENTIAL_TRIP := FALSE;
   GEN_6_BREAKER_TRIP := FALSE;
   Spare_3_201_3 := FALSE;
   GEN_6_PMA_71_FAULT := FALSE;
   GEN_6_W_LEAK_AIR_COOL := FALSE;
   Spare_3_201_6 := FALSE;
   Spare_3_201_7 := FALSE;
   GEN_6_PMA_71_STATUS := W#16#0;
   Spare_3_204_0 := FALSE;
   Spare_3_204_1 := FALSE;
   Spare_3_204_2 := FALSE;
   Spare_3_204_3 := FALSE;
   Spare_3_204_4 := FALSE;
   Spare_3_204_5 := FALSE;
   Spare_3_204_6 := FALSE;
   Spare_3_204_7 := FALSE;
   Spare_3_205_0 := FALSE;
   Spare_3_205_1 := FALSE;
   Spare_3_205_2 := FALSE;
   Spare_3_205_3 := FALSE;
   Spare_3_205_4 := FALSE;
   Spare_3_205_5 := FALSE;
   Spare_3_205_6 := FALSE;
   Spare_3_205_7 := FALSE;
   Spare_3_206_0 := FALSE;
   Spare_3_206_1 := FALSE;
   Spare_3_206_2 := FALSE;
   Spare_3_206_3 := FALSE;
   Spare_3_206_4 := FALSE;
   Spare_3_206_5 := FALSE;
   Spare_3_206_6 := FALSE;
   Spare_3_206_7 := FALSE;
   Spare_3_207_0 := FALSE;
   Spare_3_207_1 := FALSE;
   Spare_3_207_2 := FALSE;
   Spare_3_207_3 := FALSE;
   Spare_3_207_4 := FALSE;
   Spare_3_207_5 := FALSE;
   Spare_3_207_6 := FALSE;
   Spare_3_207_7 := FALSE;
   Spare_3_208_0 := FALSE;
   Spare_3_208_1 := FALSE;
   Spare_3_208_2 := FALSE;
   Spare_3_208_3 := FALSE;
   Spare_3_208_4 := FALSE;
   Spare_3_208_5 := FALSE;
   Spare_3_208_6 := FALSE;
   Spare_3_208_7 := FALSE;
   Spare_3_209_0 := FALSE;
   Spare_3_209_1 := FALSE;
   Spare_3_209_2 := FALSE;
   Spare_3_209_3 := FALSE;
   Spare_3_209_4 := FALSE;
   Spare_3_209_5 := FALSE;
   Spare_3_209_6 := FALSE;
   Spare_3_209_7 := FALSE;
   Spare_3_210 := 0;
   Spare_3_212 := 0;
   Spare_3_214 := 0;
   Spare_3_216 := 0;
   Spare_3_218 := 0;
   Spare_3_220 := 0;
   Spare_3_222 := 0;
   Spare_3_224 := 0;
   Spare_3_226 := 0;
   Spare_3_228 := 0;
   Spare_3_230 := 0;
   Spare_3_232 := 0;
   Spare_3_234 := 0;
   PacketNo3B := B#16#0;
   TelegramNo3B := B#16#0;
   PacketNo4 := B#16#0;
   TelegramNo4 := B#16#0;
   TelegramLength4 := W#16#0;
   DG_7_ENG_COOL_LVL := FALSE;
   DG_7_ENG_LO_PRESS := FALSE;
   DG_7_FO_FLT_DIFF_PR := FALSE;
   DG_7_LO_FLT_DIFF_PR := FALSE;
   DG_7_ENG_CRK_CASE_PR := FALSE;
   DG_7_MAR_GEAR_OIL_PR := FALSE;
   DG_7_ENG_JACK_WT_TEMP_HI := FALSE;
   DG_7_ENG_JACK_WT_TEMP_LO := FALSE;
   DG_7_ENG_EXH_GAS_TEMP := FALSE;
   DG_7_ENG_AFT_COOL_TEMP := FALSE;
   DG_7_MAR_GEAR_OIL_TEMP := FALSE;
   DG_7_ENG_OVERSPEED := FALSE;
   DG_7_EL_FUEL_INJ := FALSE;
   DG_7_ENG_AIR_RESTR := FALSE;
   DG_7_SYMMETRIZATION := FALSE;
   Spare_4_5_7 := FALSE;
   Spare_4_6_0 := FALSE;
   Spare_4_6_1 := FALSE;
   Spare_4_6_2 := FALSE;
   Spare_4_6_3 := FALSE;
   Spare_4_6_4 := FALSE;
   Spare_4_6_5 := FALSE;
   Spare_4_6_6 := FALSE;
   Spare_4_6_7 := FALSE;
   Spare_4_7_0 := FALSE;
   Spare_4_7_1 := FALSE;
   Spare_4_7_2 := FALSE;
   Spare_4_7_3 := FALSE;
   Spare_4_7_4 := FALSE;
   Spare_4_7_5 := FALSE;
   Spare_4_7_6 := FALSE;
   Spare_4_7_7 := FALSE;
   Spare_4_8 := 0;
   Spare_4_10 := 0;
   Spare_4_12 := 0;
   Spare_4_14 := 0;
   Spare_4_16 := 0;
   Spare_4_18 := 0;
   Spare_4_20 := 0;
   Spare_4_22 := 0;
   Spare_4_24 := 0;
   Spare_4_26 := 0;
   Spare_4_28 := 0;
   Spare_4_30 := 0;
   DG_7_EXH_GAS_CYL_01_TEMP := 0;
   DG_7_EXH_GAS_CYL_02_TEMP := 0;
   DG_7_EXH_GAS_CYL_03_TEMP := 0;
   DG_7_EXH_GAS_CYL_04_TEMP := 0;
   DG_7_EXH_GAS_CYL_05_TEMP := 0;
   DG_7_EXH_GAS_CYL_06_TEMP := 0;
   DG_7_EXH_GAS_CYL_07_TEMP := 0;
   DG_7_EXH_GAS_CYL_08_TEMP := 0;
   DG_7_EXH_GAS_CYL_09_TEMP := 0;
   DG_7_EXH_GAS_CYL_10_TEMP := 0;
   DG_7_EXH_GAS_CYL_11_TEMP := 0;
   DG_7_EXH_GAS_CYL_12_TEMP := 0;
   DG_7_EXH_GAS_CYL_13_TEMP := 0;
   DG_7_EXH_GAS_CYL_14_TEMP := 0;
   DG_7_EXH_GAS_CYL_15_TEMP := 0;
   DG_7_EXH_GAS_CYL_16_TEMP := 0;
   DG_7_EXH_CYL_TEMP_MEAN := 0;
   DG_7_EXH_GAS_TEMP_COMP := 0;
   DG_8_ENG_COOL_LVL := FALSE;
   DG_8_ENG_LO_PRESS := FALSE;
   DG_8_FO_FLT_DIFF_PR := FALSE;
   DG_8_LO_FLT_DIFF_PR := FALSE;
   DG_8_ENG_CRK_CASE_PR := FALSE;
   DG_8_MAR_GEAR_OIL_PR := FALSE;
   DG_8_ENG_JACK_WT_TEMP_HI := FALSE;
   DG_8_ENG_JACK_WT_TEMP_LO := FALSE;
   DG_8_ENG_EXH_GAS_TEMP := FALSE;
   DG_8_ENG_AFT_COOL_TEMP := FALSE;
   DG_8_MAR_GEAR_OIL_TEMP := FALSE;
   DG_8_ENG_OVERSPEED := FALSE;
   DG_8_EL_FUEL_INJ := FALSE;
   DG_8_ENG_AIR_RESTR := FALSE;
   DG_8_SYMMETRIZATION := FALSE;
   Spare_4_69_7 := FALSE;
   Spare_4_70_0 := FALSE;
   Spare_4_70_1 := FALSE;
   Spare_4_70_2 := FALSE;
   Spare_4_70_3 := FALSE;
   Spare_4_70_4 := FALSE;
   Spare_4_70_5 := FALSE;
   Spare_4_70_6 := FALSE;
   Spare_4_70_7 := FALSE;
   Spare_4_71_0 := FALSE;
   Spare_4_71_1 := FALSE;
   Spare_4_71_2 := FALSE;
   Spare_4_71_3 := FALSE;
   Spare_4_71_4 := FALSE;
   Spare_4_71_5 := FALSE;
   Spare_4_71_6 := FALSE;
   Spare_4_71_7 := FALSE;
   Spare_4_72 := 0;
   Spare_4_74 := 0;
   Spare_4_76 := 0;
   Spare_4_78 := 0;
   Spare_4_80 := 0;
   Spare_4_82 := 0;
   Spare_4_84 := 0;
   Spare_4_86 := 0;
   Spare_4_88 := 0;
   Spare_4_90 := 0;
   Spare_4_92 := 0;
   Spare_4_94 := 0;
   DG_8_EXH_GAS_CYL_01_TEMP := 0;
   DG_8_EXH_GAS_CYL_02_TEMP := 0;
   DG_8_EXH_GAS_CYL_03_TEMP := 0;
   DG_8_EXH_GAS_CYL_04_TEMP := 0;
   DG_8_EXH_GAS_CYL_05_TEMP := 0;
   DG_8_EXH_GAS_CYL_06_TEMP := 0;
   DG_8_EXH_GAS_CYL_07_TEMP := 0;
   DG_8_EXH_GAS_CYL_08_TEMP := 0;
   DG_8_EXH_GAS_CYL_09_TEMP := 0;
   DG_8_EXH_GAS_CYL_10_TEMP := 0;
   DG_8_EXH_GAS_CYL_11_TEMP := 0;
   DG_8_EXH_GAS_CYL_12_TEMP := 0;
   DG_8_EXH_GAS_CYL_13_TEMP := 0;
   DG_8_EXH_GAS_CYL_14_TEMP := 0;
   DG_8_EXH_GAS_CYL_15_TEMP := 0;
   DG_8_EXH_GAS_CYL_16_TEMP := 0;
   DG_8_EXH_CYL_TEMP_MEAN := 0;
   DG_8_EXH_GAS_TEMP_COMP := 0;
   GEN_7_VOLTAGE_L1_L2 := 0;
   GEN_7_VOLTAGE_L1_L3 := 0;
   GEN_7_VOLTAGE_L2_L3 := 0;
   GEN_7_CURRENT_L1_L2 := 0;
   GEN_7_CURRENT_L1_L3 := 0;
   GEN_7_CURRENT_L2_L3 := 0;
   GEN_7_ACTIVE_POWER := 0;
   GEN_7_POWER_FACTOR := 0;
   GEN_7_REACTIVE_POWER := 0;
   GEN_7_WDG_TEMP_L1 := 0;
   GEN_7_WDG_TEMP_L2 := 0;
   GEN_7_WDG_TEMP_L3 := 0;
   GEN_7_BEAR_TEMP_DRIVEEND := 0;
   GEN_7_BEAR_TEMP_NONDRIVE := 0;
   GEN_7_COOL_AIR_TEMP := 0;
   GEN_7_COOL_WATER_TEMP := 0;
   GEN_7_MCB_STATUS := FALSE;
   GEN_7_MCB_SEC_TO_GND := FALSE;
   GEN_7_Spare := FALSE;
   GEN_7_OVER_CURRENT_TRIP := FALSE;
   GEN_7_REVERSE_POWER_TRIP := FALSE;
   GEN_7_SHORT_CIRCUIT_TRIP := FALSE;
   GEN_7_Spare2 := FALSE;
   GEN_7_DIFF_PROT_TRIP := FALSE;
   Spare_4_165_0 := FALSE;
   GEN_7_PREFERENTIAL_TRIP := FALSE;
   GEN_7_BREAKER_TRIP := FALSE;
   Spare_4_165_3 := FALSE;
   GEN_7_PMA_71_FAULT := FALSE;
   GEN_7_W_LEAK_AIR_COOL := FALSE;
   Spare_4_165_6 := FALSE;
   Spare_4_165_7 := FALSE;
   GEN_7_PMA_71_STATUS := W#16#0;
   GEN_8_VOLTAGE_L1_L2 := 0;
   GEN_8_VOLTAGE_L1_L3 := 0;
   GEN_8_VOLTAGE_L2_L3 := 0;
   GEN_8_CURRENT_L1_L2 := 0;
   GEN_8_CURRENT_L1_L3 := 0;
   GEN_8_CURRENT_L2_L3 := 0;
   GEN_8_ACTIVE_POWER := 0;
   GEN_8_POWER_FACTOR := 0;
   GEN_8_REACTIVE_POWER := 0;
   GEN_8_WDG_TEMP_L1 := 0;
   GEN_8_WDG_TEMP_L2 := 0;
   GEN_8_WDG_TEMP_L3 := 0;
   GEN_8_BEAR_TEMP_DRIVEEND := 0;
   GEN_8_BEAR_TEMP_NONDRIVE := 0;
   GEN_8_COOL_AIR_TEMP := 0;
   GEN_8_COOL_WATER_TEMP := 0;
   GEN_8_MCB_STATUS := FALSE;
   GEN_8_MCB_SEC_TO_GND := FALSE;
   GEN_8_Spare := FALSE;
   GEN_8_OVER_CURRENT_TRIP := FALSE;
   GEN_8_REVERSE_POWER_TRIP := FALSE;
   GEN_8_SHORT_CIRCUIT_TRIP := FALSE;
   GEN_8_Spare2 := FALSE;
   GEN_8_DIFF_PROT_TRIP := FALSE;
   Spare_4_201_0 := FALSE;
   GEN_8_PREFERENTIAL_TRIP := FALSE;
   GEN_8_BREAKER_TRIP := FALSE;
   Spare_4_201_3 := FALSE;
   GEN_8_PMA_71_FAULT := FALSE;
   GEN_8_W_LEAK_AIR_COOL := FALSE;
   Spare_4_201_6 := FALSE;
   Spare_4_201_7 := FALSE;
   GEN_8_PMA_71_STATUS := W#16#0;
   Spare_4_204_0 := FALSE;
   Spare_4_204_1 := FALSE;
   Spare_4_204_2 := FALSE;
   Spare_4_204_3 := FALSE;
   Spare_4_204_4 := FALSE;
   Spare_4_204_5 := FALSE;
   Spare_4_204_6 := FALSE;
   Spare_4_204_7 := FALSE;
   Spare_4_205_0 := FALSE;
   Spare_4_205_1 := FALSE;
   Spare_4_205_2 := FALSE;
   Spare_4_205_3 := FALSE;
   Spare_4_205_4 := FALSE;
   Spare_4_205_5 := FALSE;
   Spare_4_205_6 := FALSE;
   Spare_4_205_7 := FALSE;
   Spare_4_206_0 := FALSE;
   Spare_4_206_1 := FALSE;
   Spare_4_206_2 := FALSE;
   Spare_4_206_3 := FALSE;
   Spare_4_206_4 := FALSE;
   Spare_4_206_5 := FALSE;
   Spare_4_206_6 := FALSE;
   Spare_4_206_7 := FALSE;
   Spare_4_207_0 := FALSE;
   Spare_4_207_1 := FALSE;
   Spare_4_207_2 := FALSE;
   Spare_4_207_3 := FALSE;
   Spare_4_207_4 := FALSE;
   Spare_4_207_5 := FALSE;
   Spare_4_207_6 := FALSE;
   Spare_4_207_7 := FALSE;
   Spare_4_208_0 := FALSE;
   Spare_4_208_1 := FALSE;
   Spare_4_208_2 := FALSE;
   Spare_4_208_3 := FALSE;
   Spare_4_208_4 := FALSE;
   Spare_4_208_5 := FALSE;
   Spare_4_208_6 := FALSE;
   Spare_4_208_7 := FALSE;
   Spare_4_209_0 := FALSE;
   Spare_4_209_1 := FALSE;
   Spare_4_209_2 := FALSE;
   Spare_4_209_3 := FALSE;
   Spare_4_209_4 := FALSE;
   Spare_4_209_5 := FALSE;
   Spare_4_209_6 := FALSE;
   Spare_4_209_7 := FALSE;
   Spare_4_210 := 0;
   Spare_4_212 := 0;
   Spare_4_214 := 0;
   Spare_4_216 := 0;
   Spare_4_218 := 0;
   Spare_4_220 := 0;
   Spare_4_222 := 0;
   Spare_4_224 := 0;
   Spare_4_226 := 0;
   Spare_4_228 := 0;
   Spare_4_230 := 0;
   Spare_4_232 := 0;
   Spare_4_234 := 0;
   PacketNo4B := B#16#0;
   TelegramNo4B := B#16#0;
   PacketNo5 := B#16#0;
   TelegramNo5 := B#16#0;
   TelegramLength5 := W#16#0;
   DG_9_ENG_COOL_LVL := FALSE;
   DG_9_ENG_LO_PRESS := FALSE;
   DG_9_FO_FLT_DIFF_PR := FALSE;
   DG_9_LO_FLT_DIFF_PR := FALSE;
   DG_9_ENG_CRK_CASE_PR := FALSE;
   DG_9_MAR_GEAR_OIL_PR := FALSE;
   DG_9_ENG_JACK_WT_TEMP_HI := FALSE;
   DG_9_ENG_JACK_WT_TEMP_LO := FALSE;
   DG_9_ENG_EXH_GAS_TEMP := FALSE;
   DG_9_ENG_AFT_COOL_TEMP := FALSE;
   DG_9_MAR_GEAR_OIL_TEMP := FALSE;
   DG_9_ENG_OVERSPEED := FALSE;
   DG_9_EL_FUEL_INJ := FALSE;
   DG_9_ENG_AIR_RESTR := FALSE;
   DG_9_SYMMETRIZATION := FALSE;
   Spare_5_5_7 := FALSE;
   Spare_5_6_0 := FALSE;
   Spare_5_6_1 := FALSE;
   Spare_5_6_2 := FALSE;
   Spare_5_6_3 := FALSE;
   Spare_5_6_4 := FALSE;
   Spare_5_6_5 := FALSE;
   Spare_5_6_6 := FALSE;
   Spare_5_6_7 := FALSE;
   Spare_5_7_0 := FALSE;
   Spare_5_7_1 := FALSE;
   Spare_5_7_2 := FALSE;
   Spare_5_7_3 := FALSE;
   Spare_5_7_4 := FALSE;
   Spare_5_7_5 := FALSE;
   Spare_5_7_6 := FALSE;
   Spare_5_7_7 := FALSE;
   Spare_5_8 := 0;
   Spare_5_10 := 0;
   Spare_5_12 := 0;
   Spare_5_14 := 0;
   Spare_5_16 := 0;
   Spare_5_18 := 0;
   Spare_5_20 := 0;
   Spare_5_22 := 0;
   Spare_5_24 := 0;
   Spare_5_26 := 0;
   Spare_5_28 := 0;
   Spare_5_30 := 0;
   DG_9_EXH_GAS_CYL_01_TEMP := 0;
   DG_9_EXH_GAS_CYL_02_TEMP := 0;
   DG_9_EXH_GAS_CYL_03_TEMP := 0;
   DG_9_EXH_GAS_CYL_04_TEMP := 0;
   DG_9_EXH_GAS_CYL_05_TEMP := 0;
   DG_9_EXH_GAS_CYL_06_TEMP := 0;
   DG_9_EXH_GAS_CYL_07_TEMP := 0;
   DG_9_EXH_GAS_CYL_08_TEMP := 0;
   DG_9_EXH_GAS_CYL_09_TEMP := 0;
   DG_9_EXH_GAS_CYL_10_TEMP := 0;
   DG_9_EXH_GAS_CYL_11_TEMP := 0;
   DG_9_EXH_GAS_CYL_12_TEMP := 0;
   DG_9_EXH_GAS_CYL_13_TEMP := 0;
   DG_9_EXH_GAS_CYL_14_TEMP := 0;
   DG_9_EXH_GAS_CYL_15_TEMP := 0;
   DG_9_EXH_GAS_CYL_16_TEMP := 0;
   DG_9_EXH_CYL_TEMP_MEAN := 0;
   DG_9_EXH_GAS_TEMP_COMP := 0;
   Spare_5_68_0 := FALSE;
   Spare_5_68_1 := FALSE;
   Spare_5_68_2 := FALSE;
   Spare_5_68_3 := FALSE;
   Spare_5_68_4 := FALSE;
   Spare_5_68_5 := FALSE;
   Spare_5_68_6 := FALSE;
   Spare_5_68_7 := FALSE;
   Spare_5_69_0 := FALSE;
   Spare_5_69_1 := FALSE;
   Spare_5_69_2 := FALSE;
   Spare_5_69_3 := FALSE;
   Spare_5_69_4 := FALSE;
   Spare_5_69_5 := FALSE;
   Spare_5_69_6 := FALSE;
   Spare_5_69_7 := FALSE;
   Spare_5_70_0 := FALSE;
   Spare_5_70_1 := FALSE;
   Spare_5_70_2 := FALSE;
   Spare_5_70_3 := FALSE;
   Spare_5_70_4 := FALSE;
   Spare_5_70_5 := FALSE;
   Spare_5_70_6 := FALSE;
   Spare_5_70_7 := FALSE;
   Spare_5_71_0 := FALSE;
   Spare_5_71_1 := FALSE;
   Spare_5_71_2 := FALSE;
   Spare_5_71_3 := FALSE;
   Spare_5_71_4 := FALSE;
   Spare_5_71_5 := FALSE;
   Spare_5_71_6 := FALSE;
   Spare_5_71_7 := FALSE;
   Spare_5_72 := 0;
   Spare_5_74 := 0;
   Spare_5_76 := 0;
   Spare_5_78 := 0;
   Spare_5_80 := 0;
   Spare_5_82 := 0;
   Spare_5_84 := 0;
   Spare_5_86 := 0;
   Spare_5_88 := 0;
   Spare_5_90 := 0;
   Spare_5_92 := 0;
   Spare_5_94 := 0;
   Spare_5_96 := 0;
   Spare_5_98 := 0;
   Spare_5_100 := 0;
   Spare_5_102 := 0;
   Spare_5_104 := 0;
   Spare_5_106 := 0;
   Spare_5_108 := 0;
   Spare_5_110 := 0;
   Spare_5_112 := 0;
   Spare_5_114 := 0;
   Spare_5_116 := 0;
   Spare_5_118 := 0;
   Spare_5_120 := 0;
   Spare_5_122 := 0;
   Spare_5_124 := 0;
   Spare_5_126 := 0;
   Spare_5_128 := 0;
   Spare_5_130 := 0;
   GEN_9_VOLTAGE_L1_L2 := 0;
   GEN_9_VOLTAGE_L1_L3 := 0;
   GEN_9_VOLTAGE_L2_L3 := 0;
   GEN_9_CURRENT_L1_L2 := 0;
   GEN_9_CURRENT_L1_L3 := 0;
   GEN_9_CURRENT_L2_L3 := 0;
   GEN_9_ACTIVE_POWER := 0;
   GEN_9_POWER_FACTOR := 0;
   GEN_9_REACTIVE_POWER := 0;
   GEN_9_WDG_TEMP_L1 := 0;
   GEN_9_WDG_TEMP_L2 := 0;
   GEN_9_WDG_TEMP_L3 := 0;
   GEN_9_BEAR_TEMP_DRIVEEND := 0;
   GEN_9_BEAR_TEMP_NONDRIVE := 0;
   GEN_9_COOL_AIR_TEMP := 0;
   GEN_9_COOL_WATER_TEMP := 0;
   GEN_9_MCB_STATUS := FALSE;
   GEN_9_MCB_SEC_TO_GND := FALSE;
   GEN_9_Spare := FALSE;
   GEN_9_OVER_CURRENT_TRIP := FALSE;
   GEN_9_REVERSE_POWER_TRIP := FALSE;
   GEN_9_SHORT_CIRCUIT_TRIP := FALSE;
   GEN_9_Spare2 := FALSE;
   GEN_9_DIFF_PROT_TRIP := FALSE;
   Spare_5_165_0 := FALSE;
   GEN_9_PREFERENTIAL_TRIP := FALSE;
   GEN_9_BREAKER_TRIP := FALSE;
   Spare_5_165_3 := FALSE;
   GEN_9_PMA_71_FAULT := FALSE;
   GEN_9_W_LEAK_AIR_COOL := FALSE;
   Spare_5_165_6 := FALSE;
   Spare_5_165_7 := FALSE;
   GEN_9_PMA_71_STATUS := W#16#0;
   Spare_5_168 := 0;
   Spare_5_170 := 0;
   Spare_5_172 := 0;
   Spare_5_174 := 0;
   Spare_5_176 := 0;
   Spare_5_178 := 0;
   Spare_5_180 := 0;
   Spare_5_182 := 0;
   Spare_5_184 := 0;
   Spare_5_186 := 0;
   Spare_5_188 := 0;
   Spare_5_190 := 0;
   Spare_5_192 := 0;
   Spare_5_194 := 0;
   Spare_5_196 := 0;
   Spare_5_198 := 0;
   Spare_5_200_0 := FALSE;
   Spare_5_200_1 := FALSE;
   Spare_5_200_2 := FALSE;
   Spare_5_200_3 := FALSE;
   Spare_5_200_4 := FALSE;
   Spare_5_200_5 := FALSE;
   Spare_5_200_6 := FALSE;
   Spare_5_200_7 := FALSE;
   Spare_5_201_0 := FALSE;
   Spare_5_201_1 := FALSE;
   Spare_5_201_2 := FALSE;
   Spare_5_201_3 := FALSE;
   Spare_5_201_4 := FALSE;
   Spare_5_201_5 := FALSE;
   Spare_5_201_6 := FALSE;
   Spare_5_201_7 := FALSE;
   Spare_5_202 := W#16#0;
   Spare_5_204_0 := FALSE;
   Spare_5_204_1 := FALSE;
   Spare_5_204_2 := FALSE;
   Spare_5_204_3 := FALSE;
   Spare_5_204_4 := FALSE;
   Spare_5_204_5 := FALSE;
   Spare_5_204_6 := FALSE;
   Spare_5_204_7 := FALSE;
   Spare_5_205_0 := FALSE;
   Spare_5_205_1 := FALSE;
   Spare_5_205_2 := FALSE;
   Spare_5_205_3 := FALSE;
   Spare_5_205_4 := FALSE;
   Spare_5_205_5 := FALSE;
   Spare_5_205_6 := FALSE;
   Spare_5_205_7 := FALSE;
   Spare_5_206_0 := FALSE;
   Spare_5_206_1 := FALSE;
   Spare_5_206_2 := FALSE;
   Spare_5_206_3 := FALSE;
   Spare_5_206_4 := FALSE;
   Spare_5_206_5 := FALSE;
   Spare_5_206_6 := FALSE;
   Spare_5_206_7 := FALSE;
   Spare_5_207_0 := FALSE;
   Spare_5_207_1 := FALSE;
   Spare_5_207_2 := FALSE;
   Spare_5_207_3 := FALSE;
   Spare_5_207_4 := FALSE;
   Spare_5_207_5 := FALSE;
   Spare_5_207_6 := FALSE;
   Spare_5_207_7 := FALSE;
   Spare_5_208_0 := FALSE;
   Spare_5_208_1 := FALSE;
   Spare_5_208_2 := FALSE;
   Spare_5_208_3 := FALSE;
   Spare_5_208_4 := FALSE;
   Spare_5_208_5 := FALSE;
   Spare_5_208_6 := FALSE;
   Spare_5_208_7 := FALSE;
   Spare_5_209_0 := FALSE;
   Spare_5_209_1 := FALSE;
   Spare_5_209_2 := FALSE;
   Spare_5_209_3 := FALSE;
   Spare_5_209_4 := FALSE;
   Spare_5_209_5 := FALSE;
   Spare_5_209_6 := FALSE;
   Spare_5_209_7 := FALSE;
   Spare_5_210 := 0;
   Spare_5_212 := 0;
   Spare_5_214 := 0;
   Spare_5_216 := 0;
   Spare_5_218 := 0;
   Spare_5_220 := 0;
   Spare_5_222 := 0;
   Spare_5_224 := 0;
   Spare_5_226 := 0;
   Spare_5_228 := 0;
   Spare_5_230 := 0;
   Spare_5_232 := 0;
   Spare_5_234 := 0;
   PacketNo5B := B#16#0;
   TelegramNo5B := B#16#0;
END_DATA_BLOCK

